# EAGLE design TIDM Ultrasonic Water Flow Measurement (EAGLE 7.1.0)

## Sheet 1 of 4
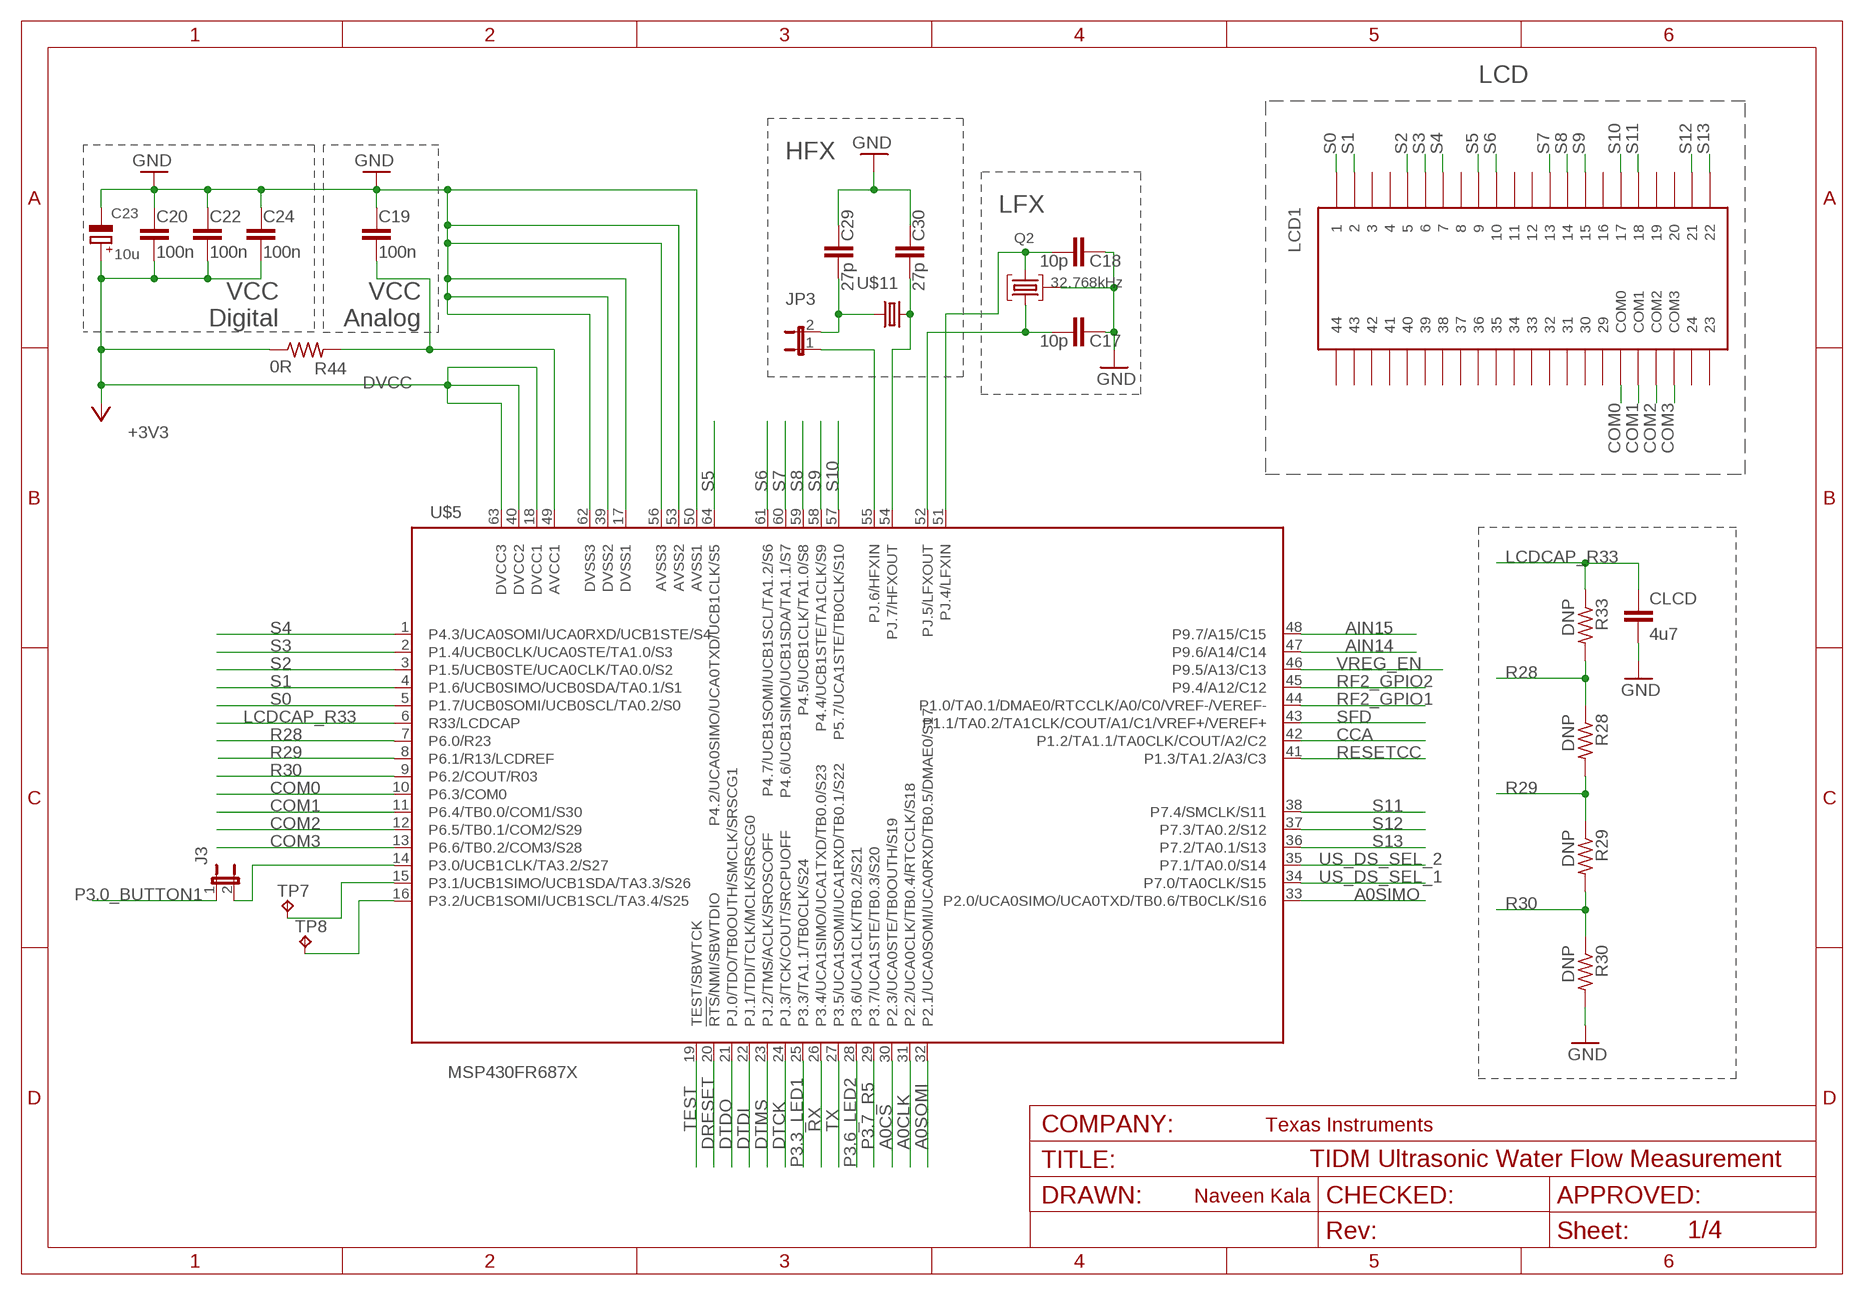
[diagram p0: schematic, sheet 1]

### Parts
C17  10p  C-EUCM0402  [0402]
C18  10p  C-EUCM0402  [0402]
C19  100n  C-EUCM0402  [0402]
C20  100n  C-EUCM0402  [0402]
C22  100n  C-EUCM0402  [0402]
C23  10u  CPOL-EUA/3216-18R  [A/3216-18R]
C24  100n  C-EUCM0402  [0402]
C29  27p  C-EUCM0402  [0402]
C30  27p  C-EUCM0402  [0402]
CLCD  4u7  CAPC0603  [0603]
J3  JP1E  [JP1]
JP3  JP1E  [JP1]
LCD1  TI_160SEG_LCD  [TI_160SEG_LCD]
Q2  32.768kHz  MS3V-T1R  [MS3V-T1R]
R28  DNP  RESR0603  [0603]
R29  DNP  RESR0603  [0603]
R30  DNP  RESR0603  [0603]
R33  DNP  RESR0603  [0603]
R44  0R  RESR0402  [0402]
TP7  TP-040  [TP-040]
TP8  TP-040  [TP-040]
U$5  MSP430FR687X  [S-PQFP-G64]
U$11  CRYSTALCTS406  [CTS406]

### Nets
A0CLK: U$5.31(P2.2/UCA0CLK/TB0.4/RTCCLK/S18) ; also sheet 2
A0CS: U$5.30(P2.3/UCA0STE/TB0OUTH/S19) ; also sheet 2
A0SIMO: U$5.33(P2.0/UCA0SIMO/UCA0TXD/TB0.6/TB0CLK/S16) ; also sheet 2,3
A0SOMI: U$5.32(P2.1/UCA0SOMI/UCA0RXD/TB0.5/DMAE0/S17) ; also sheet 2,3
AIN14: U$5.47(P9.6/A14/C14) ; also sheet 4
AIN15: U$5.48(P9.7/A15/C15) ; also sheet 4
CCA: U$5.42(P1.2/TA1.1/TA0CLK/COUT/A2/C2) ; also sheet 2
COM0: LCD1.COM0 U$5.10(P6.3/COM0)
COM1: LCD1.COM1 U$5.11(P6.4/TB0.0/COM1/S30)
COM2: LCD1.COM2 U$5.12(P6.5/TB0.1/COM2/S29)
COM3: LCD1.COM3 U$5.13(P6.6/TB0.2/COM3/S28)
DRESET: U$5.20(!RTS!/NMI/SBWTDIO) ; also sheet 3
DTCK: U$5.24(PJ.3/TCK/COUT/SRCPUOFF) ; also sheet 3
DTDI: U$5.22(PJ.1/TDI/TCLK/MCLK/SRSCG0) ; also sheet 3
DTDO: U$5.21(PJ.0/TDO/TB0OUTH/SMCLK/SRSCG1) ; also sheet 3
DTMS: U$5.23(PJ.2/TMS/ACLK/SROSCOFF) ; also sheet 3
DVCC: C20.1 C22.1 C23.+ C24.1 R44.1 U$5.18(DVCC1) U$5.40(DVCC2) U$5.63(DVCC3) ; supply symbol labelled +3V3 ; also sheet 2,3,4
GND: C17.2 C18.2 C19.2 C20.2 C22.2 C23.- C24.2 C29.2 C30.2 CLCD.2 Q2.P3(GND) R30.2 U$5.17(DVSS1) U$5.39(DVSS2) U$5.50(AVSS1) U$5.53(AVSS2) U$5.56(AVSS3) U$5.62(DVSS3) ; also sheet 2,3,4
LCDCAP_R33: CLCD.1 R33.1 U$5.6(R33/LCDCAP)
N$1: J3.2 U$5.14(P3.0/UCB1CLK/TA3.2/S27)
N$2: JP3.1 U$5.55(PJ.6/HFXIN)
N$4: TP7.1 U$5.15(P3.1/UCB1SIMO/UCB1SDA/TA3.3/S26)
N$13: C19.1 R44.2 U$5.49(AVCC1)
N$14: C30.1 U$5.54(PJ.7/HFXOUT) U$11.3
N$35: TP8.1 U$5.16(P3.2/UCB1SOMI/UCB1SCL/TA3.4/S25)
N$39: C18.1 Q2.P2 U$5.51(PJ.4/LFXIN)
N$40: C29.1 JP3.2 U$11.1
N$41: C17.1 Q2.P1 U$5.52(PJ.5/LFXOUT)
P3.0_BUTTON1: J3.1 ; also sheet 2
P3.3_LED1: U$5.25(P3.3/TA1.1/TB0CLK/S24) ; also sheet 2
P3.6_LED2: U$5.28(P3.6/UCA1CLK/TB0.2/S21) ; also sheet 2
P3.7_R5: U$5.29(P3.7/UCA1STE/TB0.3/S20) ; also sheet 4
R28: R28.1 R33.2 U$5.7(P6.0/R23)
R29: R28.2 R29.1 U$5.8(P6.1/R13/LCDREF)
R30: R29.2 R30.1 U$5.9(P6.2/COUT/R03)
RESETCC: U$5.41(P1.3/TA1.2/A3/C3) ; also sheet 2
RF2_GPIO1: U$5.44(P1.0/TA0.1/DMAE0/RTCCLK/A0/C0/VREF-/VEREF-) ; also sheet 2
RF2_GPIO2: U$5.45(P9.4/A12/C12) ; also sheet 2
RX: U$5.26(P3.4/UCA1SIMO/UCA1TXD/TB0.0/S23) ; also sheet 4
S0: LCD1.1 U$5.5(P1.7/UCB0SOMI/UCB0SCL/TA0.2/S0)
S1: LCD1.2 U$5.4(P1.6/UCB0SIMO/UCB0SDA/TA0.1/S1)
S2: LCD1.5 U$5.3(P1.5/UCB0STE/UCA0CLK/TA0.0/S2)
S3: LCD1.6 U$5.2(P1.4/UCB0CLK/UCA0STE/TA1.0/S3)
S4: LCD1.7 U$5.1(P4.3/UCA0SOMI/UCA0RXD/UCB1STE/S4)
S5: LCD1.9 U$5.64(P4.2/UCA0SIMO/UCA0TXD/UCB1CLK/S5)
S6: LCD1.10 U$5.61(P4.7/UCB1SOMI/UCB1SCL/TA1.2/S6)
S7: LCD1.13 U$5.60(P4.6/UCB1SIMO/UCB1SDA/TA1.1/S7)
S8: LCD1.14 U$5.59(P4.5/UCB1CLK/TA1.0/S8)
S9: LCD1.15 U$5.58(P4.4/UCB1STE/TA1CLK/S9)
S10: LCD1.17 U$5.57(P5.7/UCA1STE/TB0CLK/S10)
S11: LCD1.18 U$5.38(P7.4/SMCLK/S11)
S12: LCD1.21 U$5.37(P7.3/TA0.2/S12)
S13: LCD1.22 U$5.36(P7.2/TA0.1/S13)
SFD: U$5.43(P1.1/TA0.2/TA1CLK/COUT/A1/C1/VREF+/VEREF+) ; also sheet 2
TEST: U$5.19(TEST/SBWTCK) ; also sheet 3
TX: U$5.27(P3.5/UCA1SOMI/UCA1RXD/TB0.1/S22) ; also sheet 4
US_DS_SEL_1: U$5.34(P7.0/TA0CLK/S15) ; also sheet 4
US_DS_SEL_2: U$5.35(P7.1/TA0.0/S14) ; also sheet 4
VREG_EN: U$5.46(P9.5/A13/C13) ; also sheet 2
Unconnected: LCD1.3 LCD1.4 LCD1.8 LCD1.11 LCD1.12 LCD1.16 LCD1.19 LCD1.20 LCD1.23 LCD1.24 LCD1.29 LCD1.30 LCD1.31 LCD1.32 LCD1.33 LCD1.34 LCD1.35 LCD1.36 LCD1.37 LCD1.38 LCD1.39 LCD1.40 LCD1.41 LCD1.42 LCD1.43 LCD1.44

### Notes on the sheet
- LCD
- HFX
- LFX
- VCC | VCC
- Digital | Analog
- Texas Instruments
- Naveen Kala

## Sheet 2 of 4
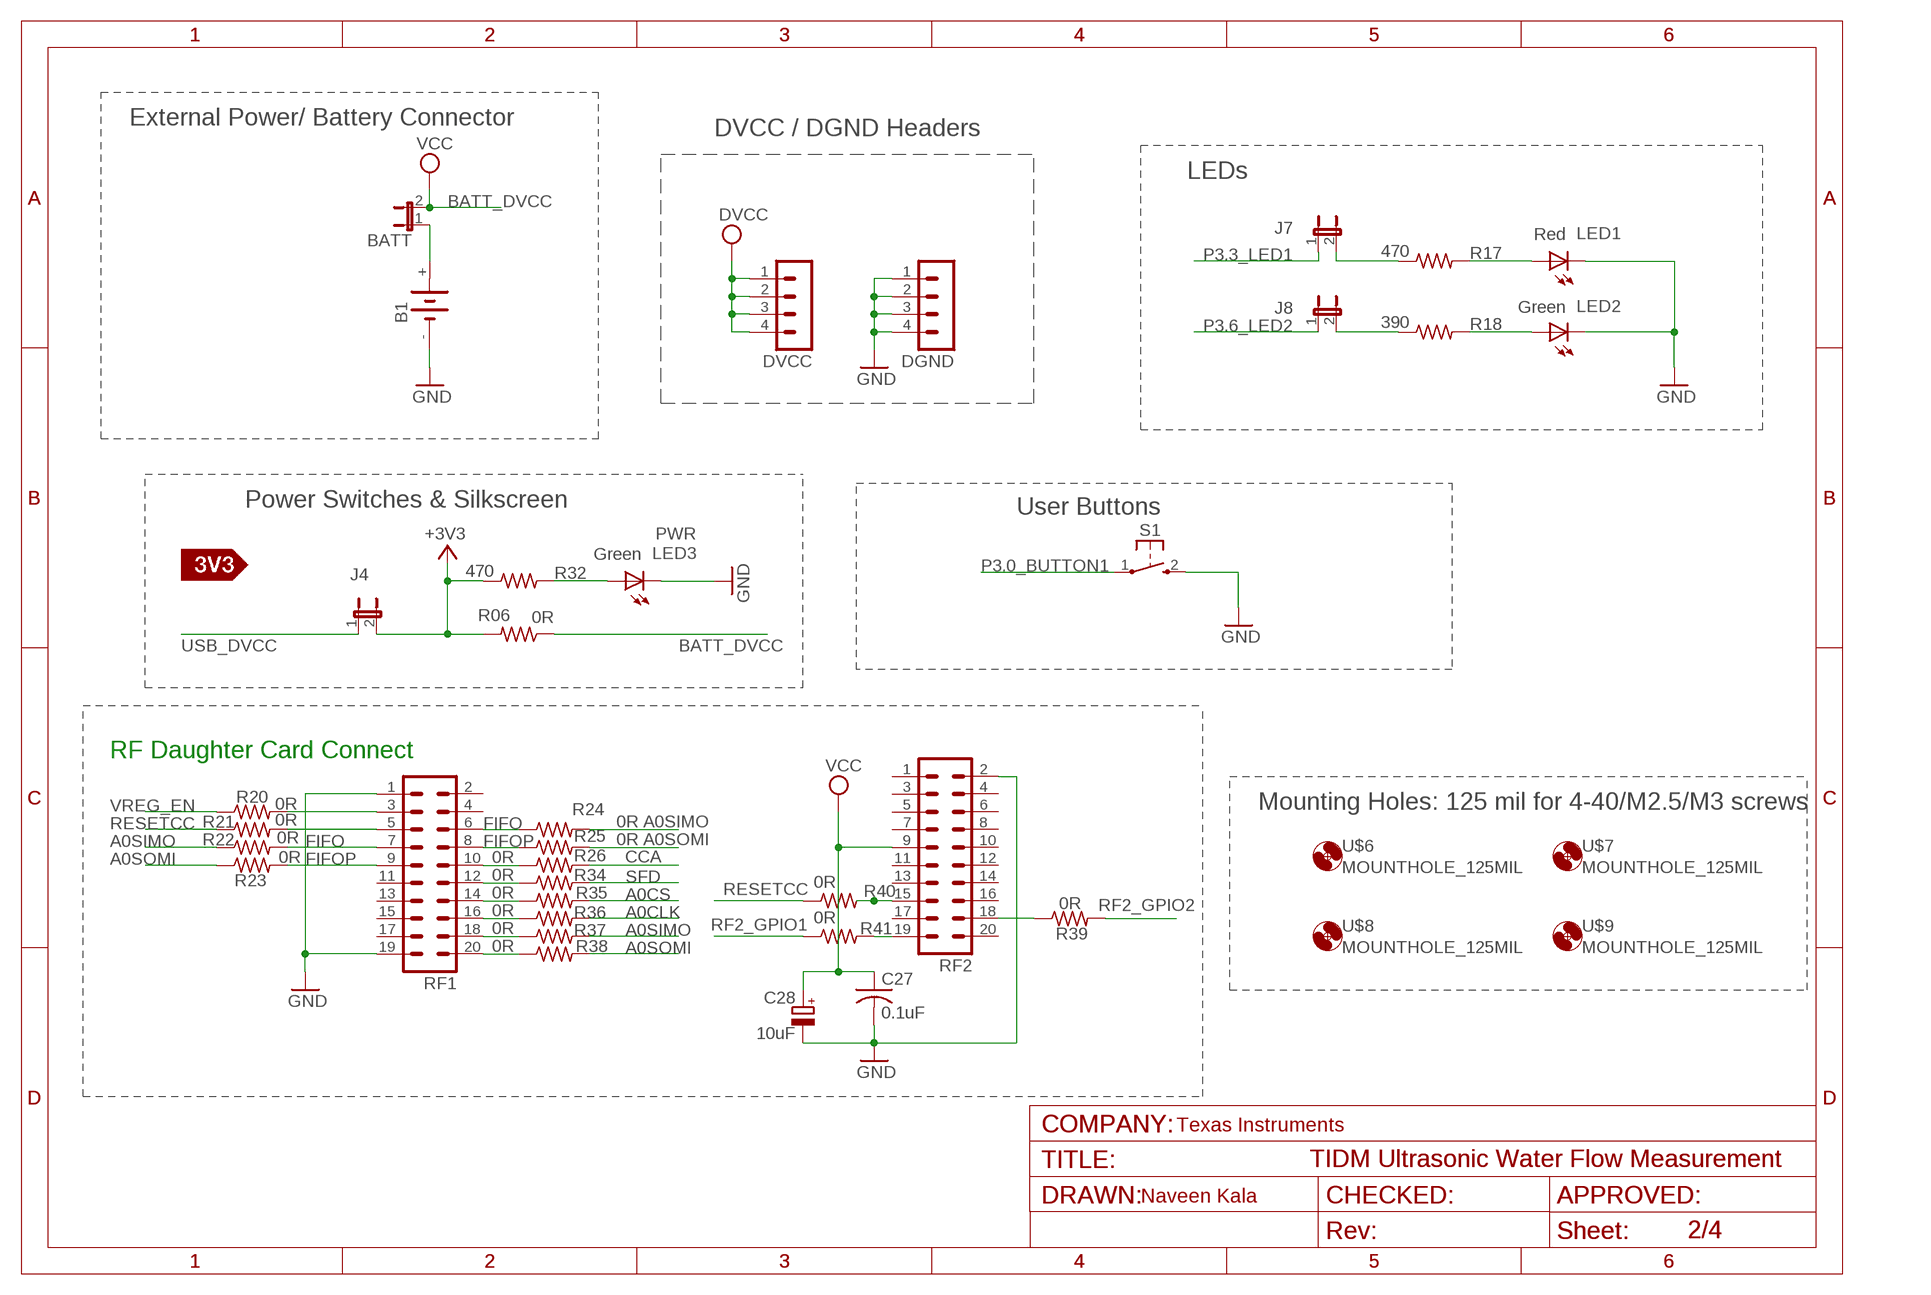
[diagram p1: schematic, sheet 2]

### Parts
B1  KS2468NO_HOLES  [KS2468_2]
BATT  JP1E  [JP1]
C27  0.1uF  C-USC0805  [C0805]
C28  10uF  CPOL-EUA/3216-18R  [A/3216-18R]
DGND  MA04-1  [MA04-1]
DVCC  MA04-1  [MA04-1]
J4  JUMPER_2.51MM  [JUMPER-2.54]
J7  JUMPER_2.51MM  [JUMPER-2.54]
J8  JUMPER_2.51MM  [JUMPER-2.54]
LED1  Red  CHIP-LED  [LED0805]
LED2  Green  CHIP-LED  [LED0805]
LED3  Green  CHIP-LED  [LED0805]
R06  0R  RESR0402  [0402]
R17  470  R-US_R0402  [R0402]
R18  390  R-US_R0402  [R0402]
R20  0R  R-US_R0603  [R0603]
R21  0R  R-US_R0603  [R0603]
R22  0R  R-US_R0603  [R0603]
R23  0R  R-US_R0603  [R0603]
R24  0R  R-US_R0603  [R0603]
R25  0R  R-US_R0603  [R0603]
R26  0R  R-US_R0603  [R0603]
R32  470  RESR0402  [0402]
R34  0R  R-US_R0603  [R0603]
R35  0R  R-US_R0603  [R0603]
R36  0R  R-US_R0603  [R0603]
R37  0R  R-US_R0603  [R0603]
R38  0R  R-US_R0603  [R0603]
R39  0R  R-US_R0603  [R0603]
R40  0R  R-US_R0603  [R0603]
R41  0R  R-US_R0603  [R0603]
RF1  TFM-110-02-SM-D-A-K  [TFM-110-02-SM-D-A-K]
RF2  TFM-110-02-SM-D-A-K  [TFM-110-02-SM-D-A-K]
S1  PB  [PBTH]
U$6  MOUNTHOLE_125MIL  [MOUNTHOLE_125MIL]
U$7  MOUNTHOLE_125MIL  [MOUNTHOLE_125MIL]
U$8  MOUNTHOLE_125MIL  [MOUNTHOLE_125MIL]
U$9  MOUNTHOLE_125MIL  [MOUNTHOLE_125MIL]
U$10  SILK_3V3_TAG  [SILK_3V3_TAG]

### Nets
$1: R20.2 RF1.3
$2: R21.2 RF1.5
A0CLK: R36.2 ; also sheet 1
A0CS: R35.2 ; also sheet 1
A0SIMO: R22.1 R24.2 R37.2 ; also sheet 1,3
A0SOMI: R23.1 R25.2 R38.2 ; also sheet 1,3
BATT_DVCC: BATT.2 R06.1 ; supply symbol labelled VCC
CCA: R26.2 ; also sheet 1
DVCC: DVCC.1 DVCC.2 DVCC.3 DVCC.4 J4.2 R06.2 R32.1 ; supply symbol labelled +3V3 ; also sheet 1,3,4
FIFO: R22.2 R24.1 RF1.6 RF1.7
FIFOP: R23.2 R25.1 RF1.8 RF1.9
GND: B1.- C27.2 C28.- DGND.1 DGND.2 DGND.3 DGND.4 LED1.C LED2.C LED3.C RF1.1 RF1.19 RF2.2 S1.2(S) ; also sheet 1,3,4
N$3: J8.2 R18.1
N$6: J7.2 R17.1
N$7: LED1.A R17.2
N$8: LED2.A R18.2
N$9: B1.+ BATT.1
N$19: R26.1 RF1.10
N$20: R34.1 RF1.12
N$23: R35.1 RF1.14
N$26: R36.1 RF1.16
N$27: R37.1 RF1.18
N$28: R38.1 RF1.20
N$29: R39.1 RF2.18
N$30: R40.2 RF2.15
N$31: R41.2 RF2.19
N$38: LED3.A R32.2
P3.0_BUTTON1: S1.1(P) ; also sheet 1
P3.3_LED1: J7.1 ; also sheet 1
P3.6_LED2: J8.1 ; also sheet 1
RESETCC: R21.1 R40.1 ; also sheet 1
RF2_GPIO1: R41.1 ; also sheet 1
RF2_GPIO2: R39.2 ; also sheet 1
SFD: R34.2 ; also sheet 1
USB_DVCC: J4.1 ; also sheet 3
VCC: C27.1 C28.+ RF2.9
VREG_EN: R20.1 ; also sheet 1
Unconnected: RF1.2 RF1.4 RF1.11 RF1.13 RF1.15 RF1.17 RF2.1 RF2.3 RF2.4 RF2.5 RF2.6 RF2.7 RF2.8 RF2.10 RF2.11 RF2.12 RF2.13 RF2.14 RF2.16 RF2.17 RF2.20

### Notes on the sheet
- External Power/ Battery Connector
- DVCC / DGND Headers
- LEDs
- Power Switches & Silkscreen
- User Buttons
- PWR
- RF Daughter Card Connect
- Mounting Holes: 125 mil for 4-40/M2.5/M3 screws
- Texas Instruments
- Naveen Kala

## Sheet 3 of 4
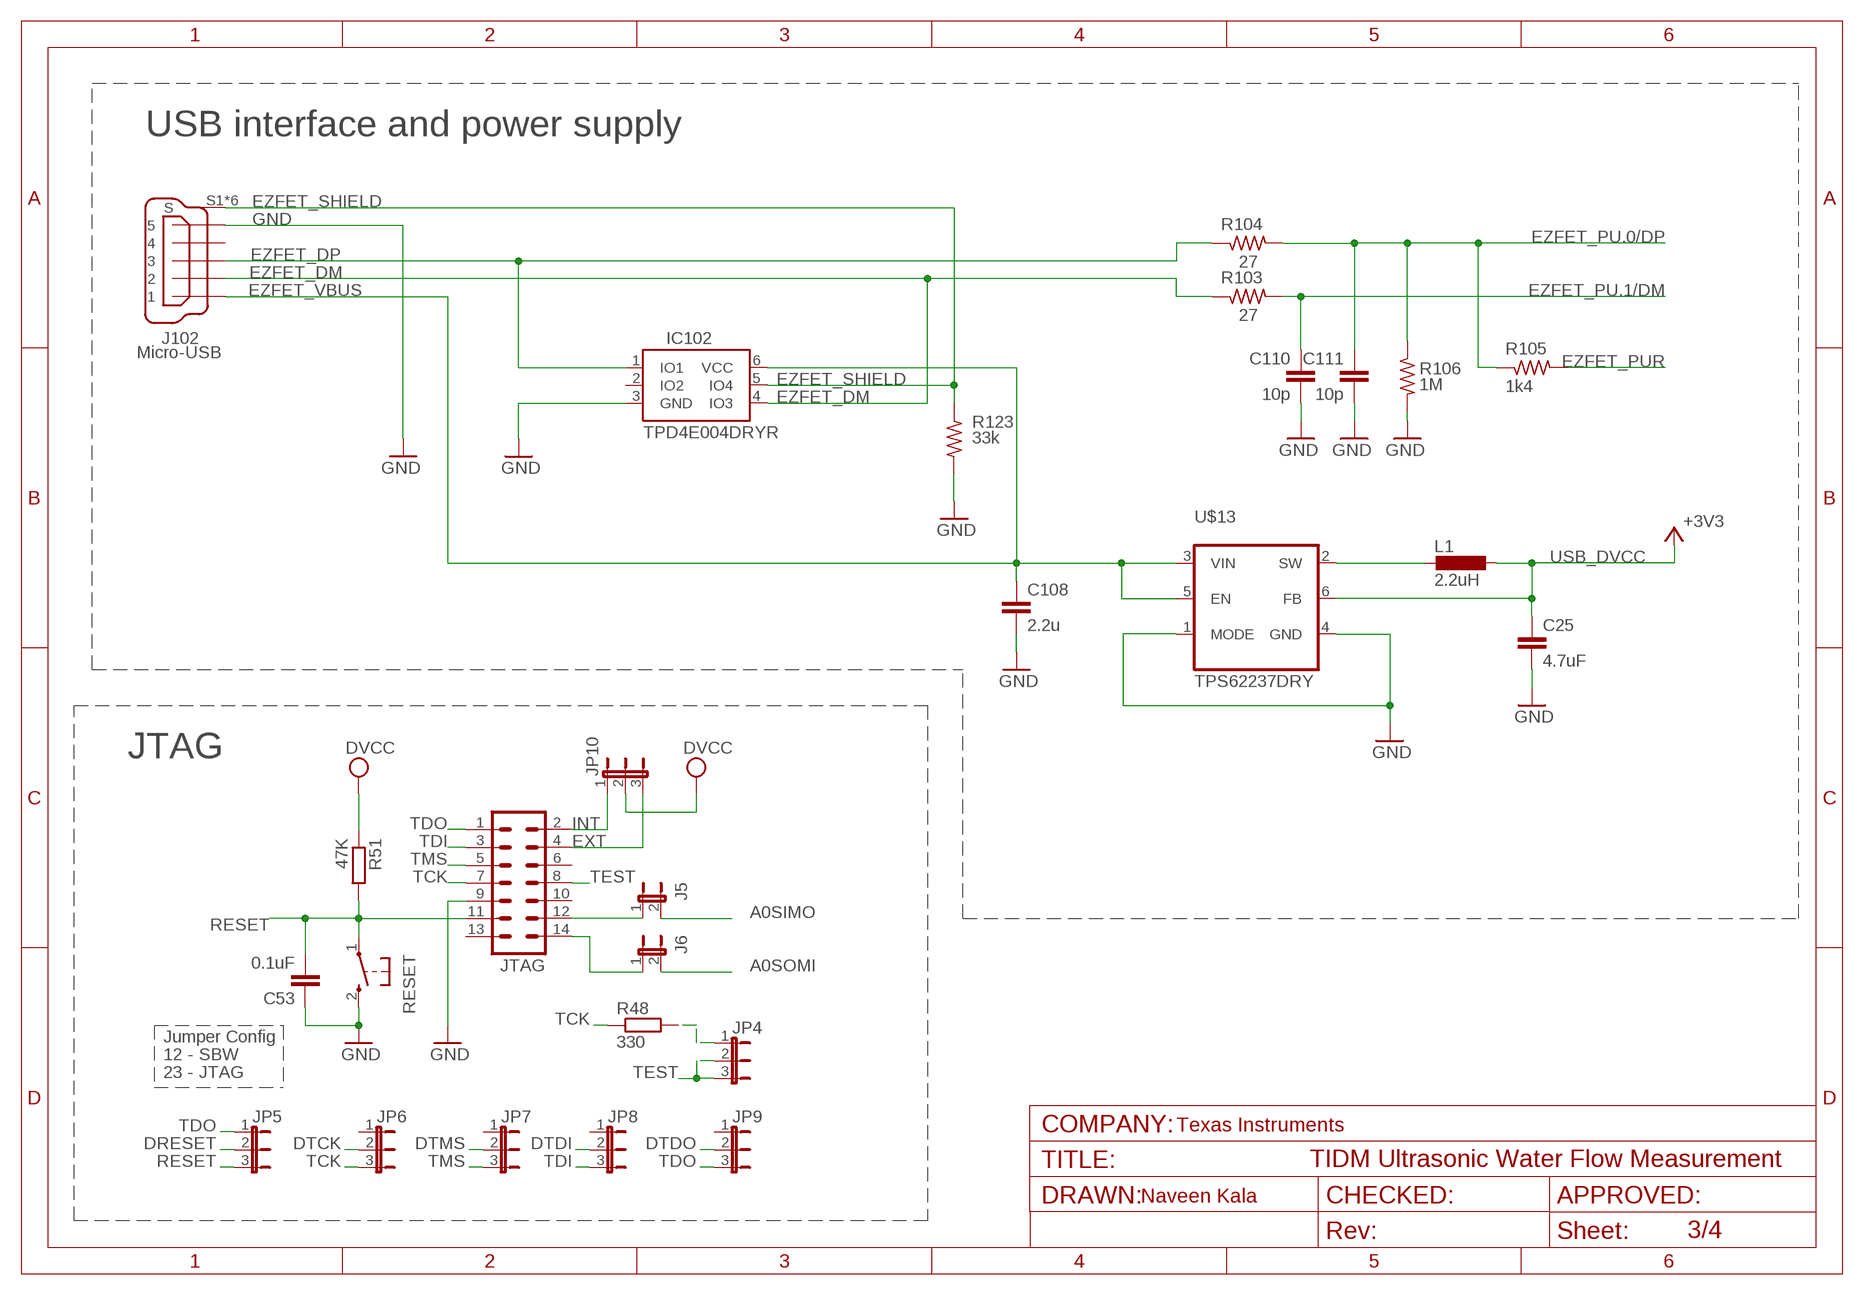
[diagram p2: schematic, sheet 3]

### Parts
C25  4.7uF  C-EUC0402  [C0402]
C53  0.1uF  C-EUC0603  [C0603]
C108  2.2u  C-EUC0603  [C0603]
C110  10p  C-EUCM0402  [0402]
C111  10p  C-EUCM0402  [0402]
IC102  TPD4E004DRYR  TPD4E004  [SON(DRY)6]
J5  JP1E  [JP1]
J6  JP1E  [JP1]
J102  Micro-USB  EZFET_MINI-USB-  [EZFET_UX62M-B-5P]
JP4  JP2E  [JP2]
JP5  JP2E  [JP2]
JP6  JP2E  [JP2]
JP7  JP2E  [JP2]
JP8  JP2E  [JP2]
JP9  JP2E  [JP2]
JP10  JP2E  [JP2]
JTAG  ML14  [ML14]
L1  2.2uH  L-EUL2012C  [L2012C]
R48  330  R-EU_R0603  [R0603]
R51  47K  R-EU_R0603  [R0603]
R103  27  RESR0402  [0402]
R104  27  RESR0402  [0402]
R105  1k4  RESR0402  [0402]
R106  1M  RESR0402  [0402]
R123  33k  RESR0402  [0402]
RESET  PB  [PBTH]
U$13  TPS62237DRY  [DRY(R-PUSON-N6)]

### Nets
A0SIMO: J5.2 ; also sheet 1,2
A0SOMI: J6.2 ; also sheet 1,2
DRESET: JP5.2 ; also sheet 1
DTCK: JP6.2 ; also sheet 1
DTDI: JP8.2 ; also sheet 1
DTDO: JP9.2 ; also sheet 1
DTMS: JP7.2 ; also sheet 1
DVCC: JP10.2 R51.1 ; also sheet 1,2,4
EXT: JP10.3 JTAG.4
EZFET_DM: IC102.4(IO3) J102.2 R103.1
EZFET_DP: IC102.1(IO1) J102.3 R104.1
EZFET_PU.0/DP: C111.1 R104.2 R105.1 R106.1
EZFET_PU.1/DM: C110.1 R103.2
EZFET_PUR: R105.2
EZFET_SHIELD: IC102.5(IO4) J102.S1(S) J102.S2(S) J102.S3(S) J102.S4(S) J102.S5(S) J102.S6(S) R123.1
EZFET_VBUS: C108.1 IC102.6(VCC) J102.1 U$13.3(VIN) U$13.5(EN)
GND: C25.2 C53.1 C108.2 C110.2 C111.2 IC102.3(GND) J102.5 JTAG.9 R106.2 R123.2 RESET.2(S) U$13.1(MODE) U$13.4(GND) ; also sheet 1,2,4
INT: JP10.1 JTAG.2
N$5: L1.2 U$13.2(SW)
N$10: JP4.1 R48.2
N$12: J6.1 JTAG.14
N$42: J5.1 JTAG.12
RESET: C53.2 JP5.3 JTAG.11 R51.2 RESET.1(P)
TCK: JP6.3 JTAG.7 R48.1
TDI: JP8.3 JTAG.3
TDO: JP5.1 JP9.3 JTAG.1
TEST: JP4.2 JP4.3 JTAG.8 ; also sheet 1
TMS: JP7.3 JTAG.5
USB_DVCC: C25.1 L1.1 U$13.6(FB) ; supply symbol labelled +3V3 ; also sheet 2
Unconnected: IC102.2(IO2) J102.4 JP6.1 JP7.1 JP8.1 JP9.1 JTAG.6 JTAG.10 JTAG.13

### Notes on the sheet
- USB interface and power supply
- JTAG
- Jumper Config
- 12 - SBW
- 23 - JTAG
- Texas Instruments
- Naveen Kala

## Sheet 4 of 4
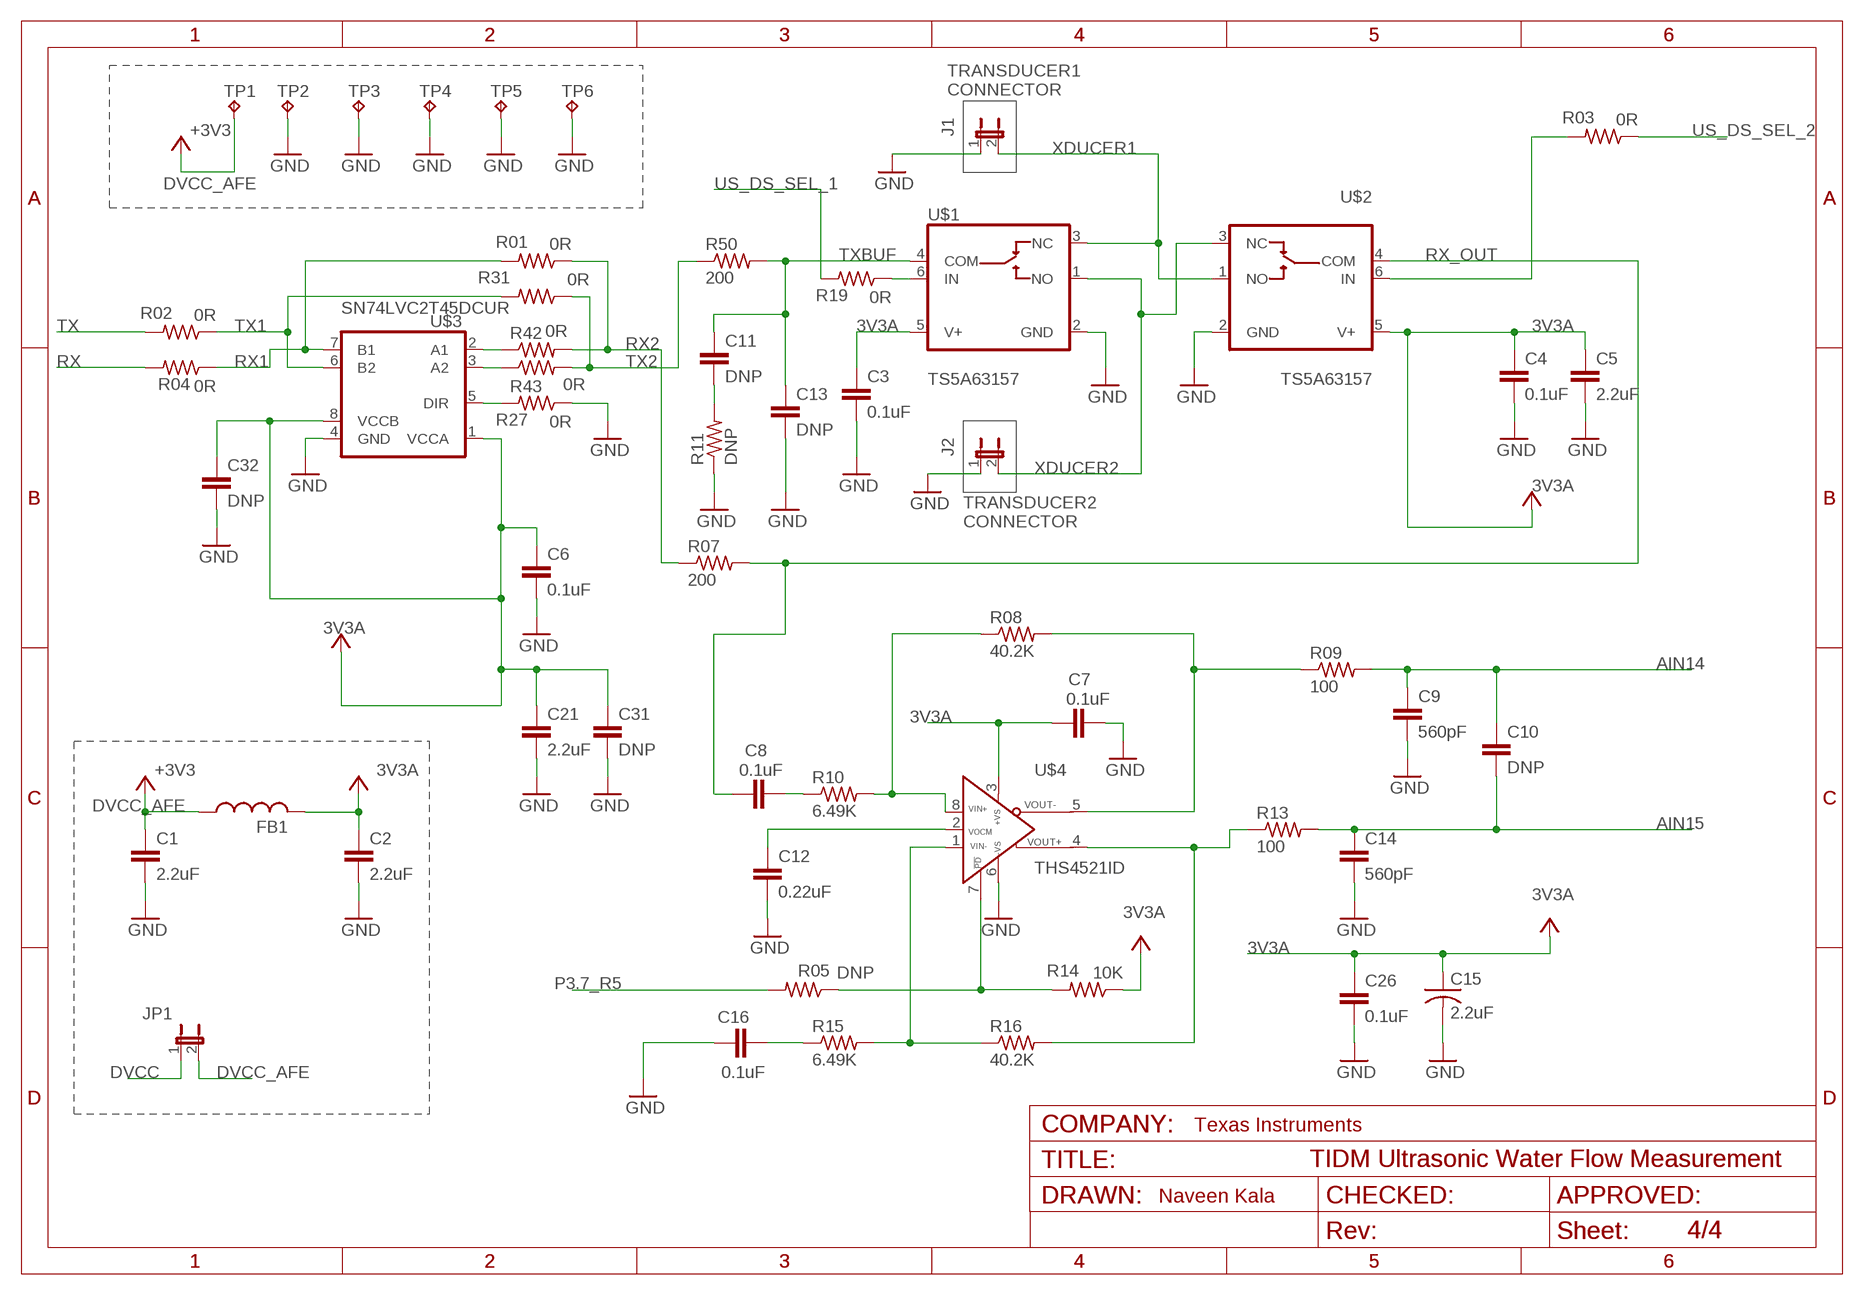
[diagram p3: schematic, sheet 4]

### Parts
C1  2.2uF  C-EUC0603  [C0603]
C2  2.2uF  C-EUC0603  [C0603]
C3  0.1uF  C-EUC0402  [C0402]
C4  0.1uF  C-EUC0402  [C0402]
C5  2.2uF  C-EUC0603  [C0603]
C6  0.1uF  C-EUC0402  [C0402]
C7  0.1uF  C-EUC0402  [C0402]
C8  0.1uF  C-EUC0603  [C0603]
C9  560pF  C-EUC0402  [C0402]
C10  DNP  C-EUC0805  [C0805@1]
C11  DNP  C-EUC0603  [C0603]
C12  0.22uF  C-EUC0402  [C0402]
C13  DNP  C-EUC0603  [C0603]
C14  560pF  C-EUC0402  [C0402]
C15  2.2uF  C-USC0603  [C0603]
C16  0.1uF  C-EUC0603  [C0603]
C21  2.2uF  C-EUC0603  [C0603]
C26  0.1uF  C-EUC0603  [C0603]
C31  DNP  C-EUC0603  [C0603]
C32  DNP  C-EUC0603  [C0603]
FB1  L-0603  [L-603]
J1  JP1E  [JP1]
J2  JP1E  [JP1]
JP1  JP1E  [JP1]
R01  0R  RESR0402  [0402]
R02  0R  RESR0402  [0402]
R03  0R  RESR0402  [0402]
R04  0R  RESR0402  [0402]
R05  DNP  RESR0402  [0402]
R07  200  R-US_R0805  [R0805]
R08  40.2K  R-US_R0805  [R0805]
R09  100  R-US_R0603  [R0603]
R10  6.49K  R-US_R0603  [R0603]
R11  DNP  R-US_R0603  [R0603]
R13  100  R-US_R0603  [R0603]
R14  10K  RESR0402  [0402]
R15  6.49K  R-US_R0603  [R0603]
R16  40.2K  R-US_R0805  [R0805]
R19  0R  RESR0402  [0402]
R27  0R  RESR0402  [0402]
R31  0R  RESR0402  [0402]
R42  0R  R-US_R0603  [R0603]
R43  0R  R-US_R0603  [R0603]
R50  200  R-US_R0805  [R0805]
TP1  TP-040  [TP-040]
TP2  TP-040  [TP-040]
TP3  TP-040  [TP-040]
TP4  TP-040  [TP-040]
TP5  TP-040  [TP-040]
TP6  TP-040  [TP-040]
U$1  TS5A63157  [DCK_R-PDSO-G6]
U$2  TS5A63157  [DCK_R-PDSO-G6]
U$3  SN74LVC2T45DCUR  [DCT(R-PDSO-G8)]
U$4  THS4521ID  [SOIC08(D-R-PDSO-G8)]

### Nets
3V3A: C2.1 C3.1 C4.1 C5.1 C6.1 C7.1 C15.1 C21.1 C26.1 C31.1 C32.1 FB1.2 R14.1 U$1.5(V+) U$2.5(V+) U$3.1(VCCA) U$3.8(VCCB) U$4.3(+VS) ; supply symbol labelled VCC
AIN14: C9.1 C10.1 R09.2 ; also sheet 1
AIN15: C10.2 C14.1 R13.2 ; also sheet 1
DIR: R27.2 U$3.5(DIR)
DVCC: JP1.1 ; also sheet 1,2,3
DVCC_AFE: C1.1 FB1.1 JP1.2 TP1.1 ; supply symbol labelled +3V3
GND: C1.2 C2.2 C3.2 C4.2 C5.2 C6.2 C7.2 C9.2 C12.2 C13.2 C14.2 C15.2 C16.1 C21.2 C26.2 C31.2 C32.2 J1.1 J2.1 R11.1 R27.1 TP2.1 TP3.1 TP4.1 TP5.1 TP6.1 U$1.2(GND) U$2.2(GND) U$3.4(GND) U$4.6(-VS) ; also sheet 1,2,3
N$11: R19.1 U$1.6(IN)
N$15: C11.2 R11.2
N$16: R03.2 U$2.6(IN)
N$17: R08.2 R09.1 U$4.5(VOUT-)
N$18: R13.1 R16.2 U$4.4(VOUT+)
N$21: R15.2 R16.1 U$4.1(VIN-)
N$22: C16.2 R15.1
N$24: R08.1 R10.2 U$4.8(VIN+)
N$25: C8.2 R10.1
N$32: R05.1 R14.2 U$4.7(!PD!)
N$33: R42.1 U$3.2(A1)
N$34: R43.1 U$3.3(A2)
P3.7_R5: R05.2 ; also sheet 1
RX: R04.2 ; also sheet 1
RX1: R01.2 R04.1 U$3.7(B1)
RX2: R01.1 R07.1 R42.2
RX_OUT: C8.1 R07.2 U$2.4(COM)
TX: R02.2 ; also sheet 1
TX1: R02.1 R31.2 U$3.6(B2)
TX2: R31.1 R43.2 R50.1
TXBUF: C11.1 C13.1 R50.2 U$1.4(COM)
US_DS_SEL_1: R19.2 ; also sheet 1
US_DS_SEL_2: R03.1 ; also sheet 1
VOCM: C12.1 U$4.2(VOCM)
XDUCER1: J1.2 U$1.3(NC) U$2.1(NO)
XDUCER2: J2.2 U$1.1(NO) U$2.3(NC)

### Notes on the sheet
- TRANSDUCER1
  CONNECTOR
- 3V3A
- TRANSDUCER2
  CONNECTOR
- 3V3A
- 3V3A
- 3V3A
- 3V3A
- Texas Instruments
- Naveen Kala

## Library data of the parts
B1 = _MSP430:KS2468
BATT J1-J3 J5 J6 JP1 JP3 = jumper:JP1E: JUMPER
C1-C14 C16-C22 C24-C26 C29-C32 C108 C110 C111 = rcl:C-EU: CAPACITOR, European symbol
C15 C27 = rcl:C-US: CAPACITOR, American symbol
C23 C28 = rcl:CPOL-EU: POLARIZED CAPACITOR, European symbol
C53 = resistor:C-EU: CAPACITOR, European symbol
CLCD = MSP430_CapResistor:CAP
DGND DVCC = custom_con-lstb:MA04-1: PIN HEADER; OC_FARNELL: unknown; OC_NEWARK: unknown
FB1 = HVK-Ultrasonic-FM:L-0603
IC102 = eZFET:TPD4E004
J4 J7 J8 = launchpad:JUMPER_2.51MM
J102 = MSP-EXP430G6021:EZFET_MINI-USB-: MINI USB Connector Source: http://www.hirose.co.jp/cataloge_hp/e24000019.pdf
JP4-JP10 = custom_jumper:JP2E: JUMPER
JTAG = con-ml:ML14: HARTING; OC_FARNELL: unknown; OC_NEWARK: unknown
L1 = rcl:L-EU: INDUCTOR, European symbol
LCD1 = Personal:TI_160SEG_LCD
LED1-LED3 = launchpad:CHIP-LED
Q2 = microcrystal:MS3V-T1R
R01-R06 R14 R19 R27-R33 R44 R103-R106 R123 = CapResistor:RES
R07-R09 R10 R11 R13 R15-R18 R20-R26 R34-R43 R50 = rcl:R-US_: RESISTOR, American symbol
R48 R51 = resistor:R-EU_: RESISTOR, European symbol
RESET S1 = electricalmeter:PB: OMRON SWITCH
RF1 RF2 = _MSP430:TFM-110-02-SM-D-A-K
TP1-TP8 = keystone:TP: TEST POINT
U$1 U$2 = HVK-Ultrasonic-FM:TS5A63157
U$3 = HVK-Ultrasonic-FM:SN74LVC2T45DCUR
U$4 = HVK-Ultrasonic-FM:THS4521ID
U$5 = HVK-Ultrasonic-FM:MSP430FR687X
U$6-U$9 = MSP-EXP432:MOUNTHOLE_125MIL
U$10 = MSP-EXP432:SILK_3V3_TAG
U$11 = crystal:CRYSTAL: CRYSTAL; OC_FARNELL: unknown; OC_NEWARK: unknown
U$13 = HVK-Ultrasonic-FM:TPS62237DRY

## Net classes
2 Power: width 0.203 mm, drill 0.305 mm, clearance 0.152 mm to class 0, clearance 0.152 mm to class 1, clearance 0.152 mm

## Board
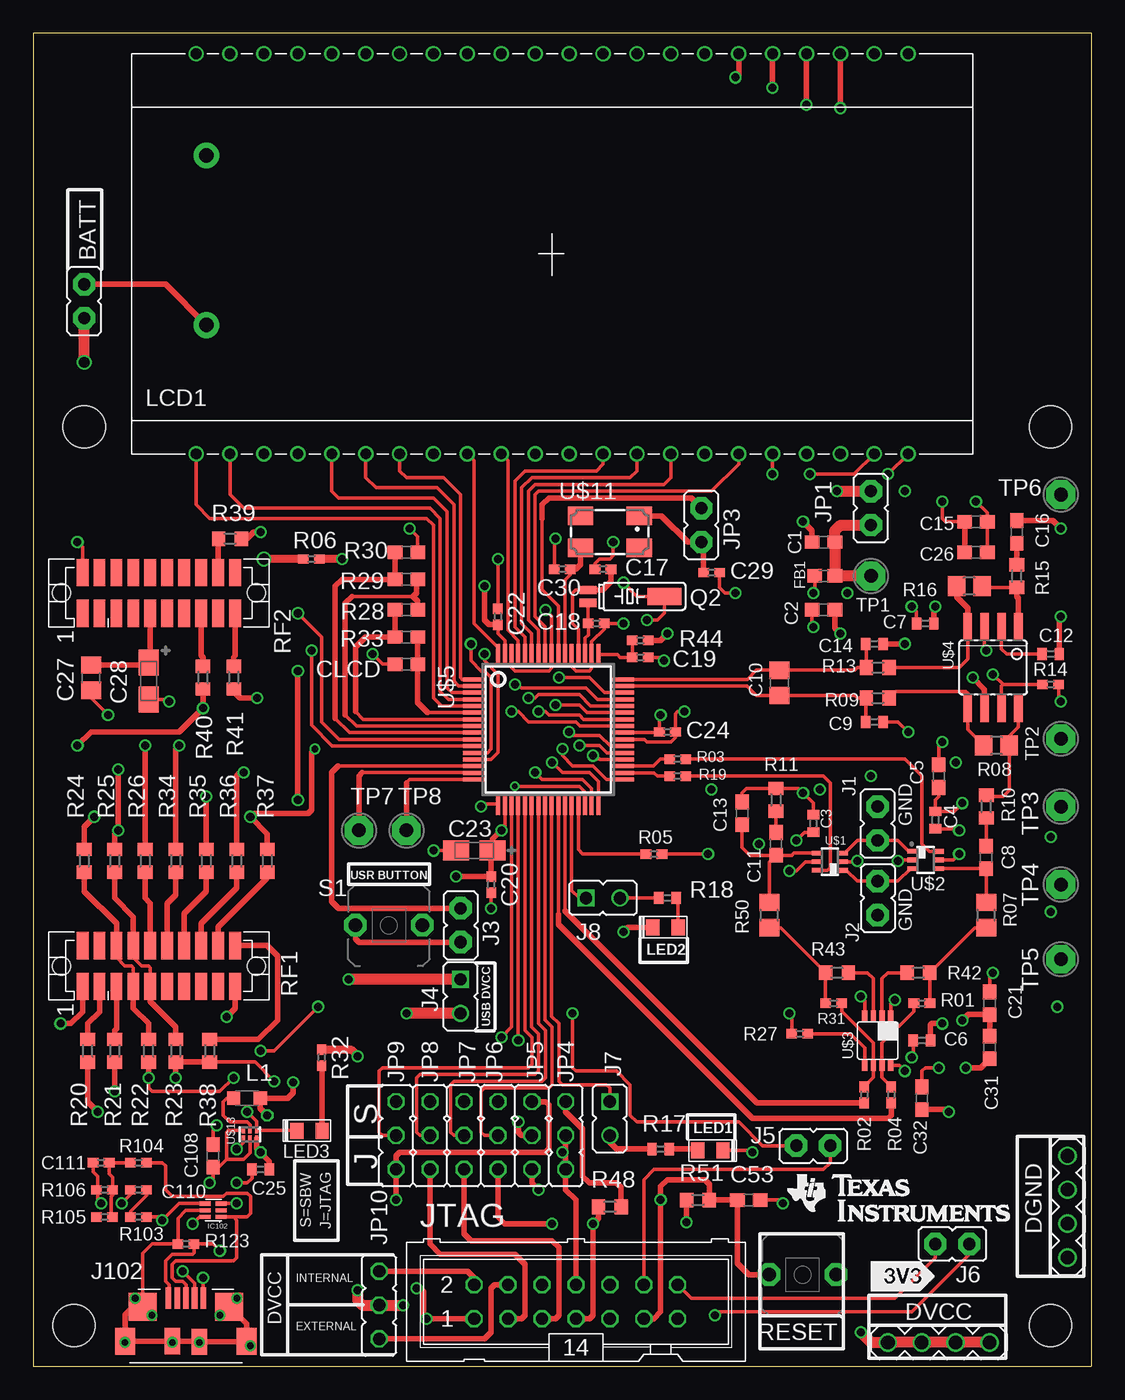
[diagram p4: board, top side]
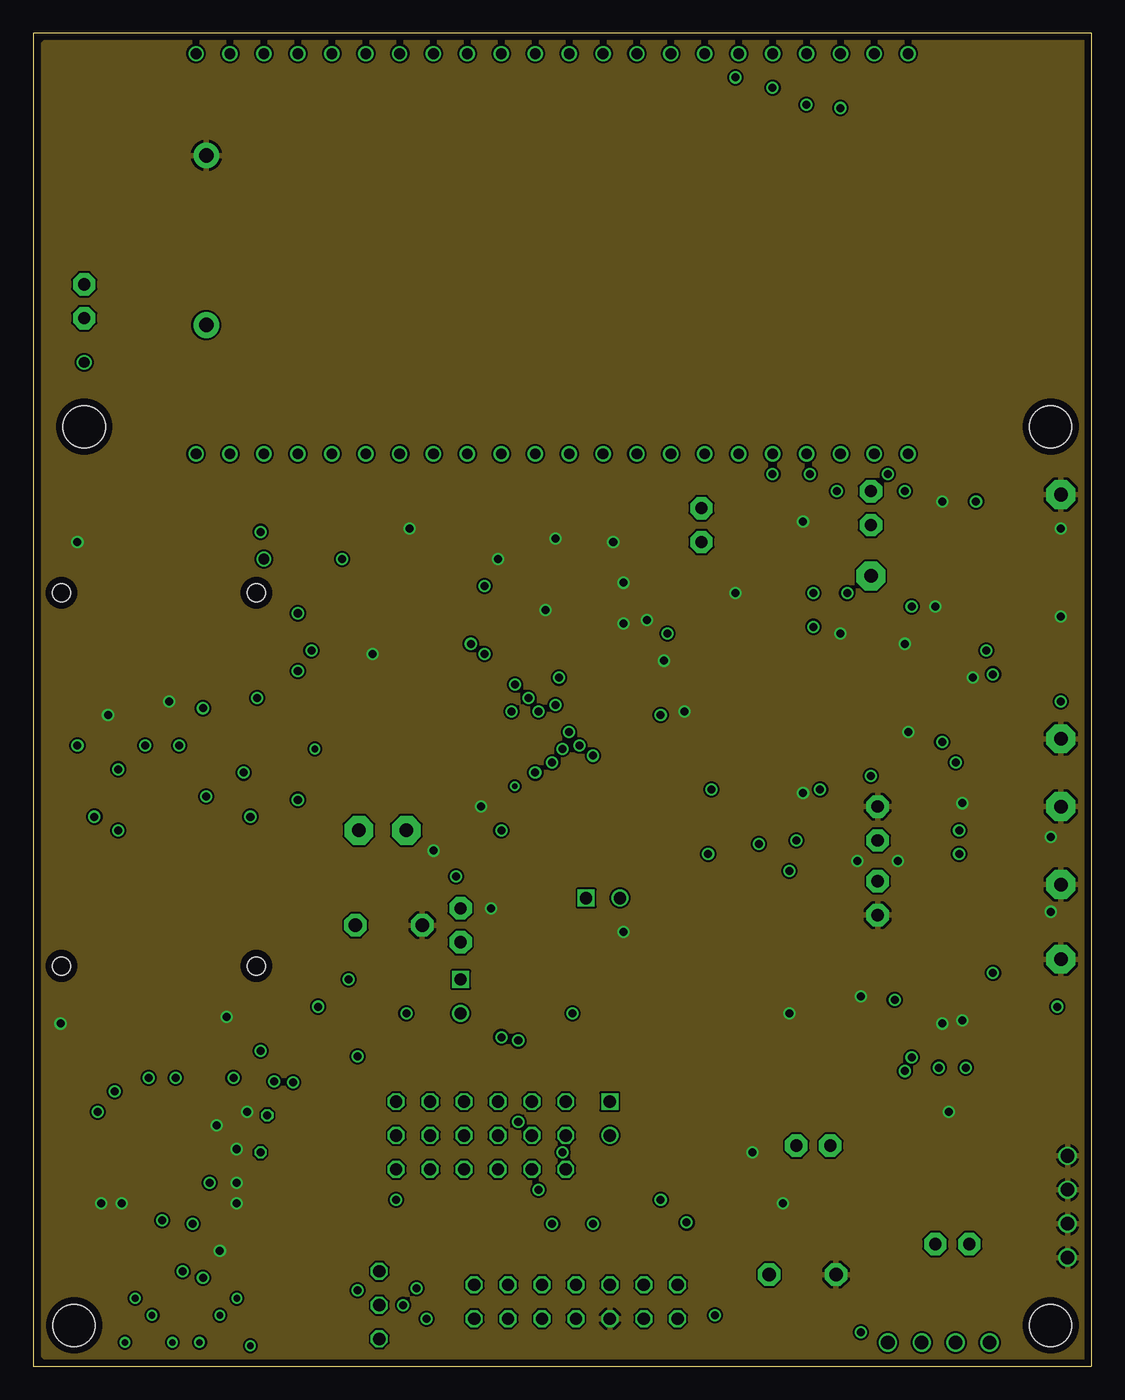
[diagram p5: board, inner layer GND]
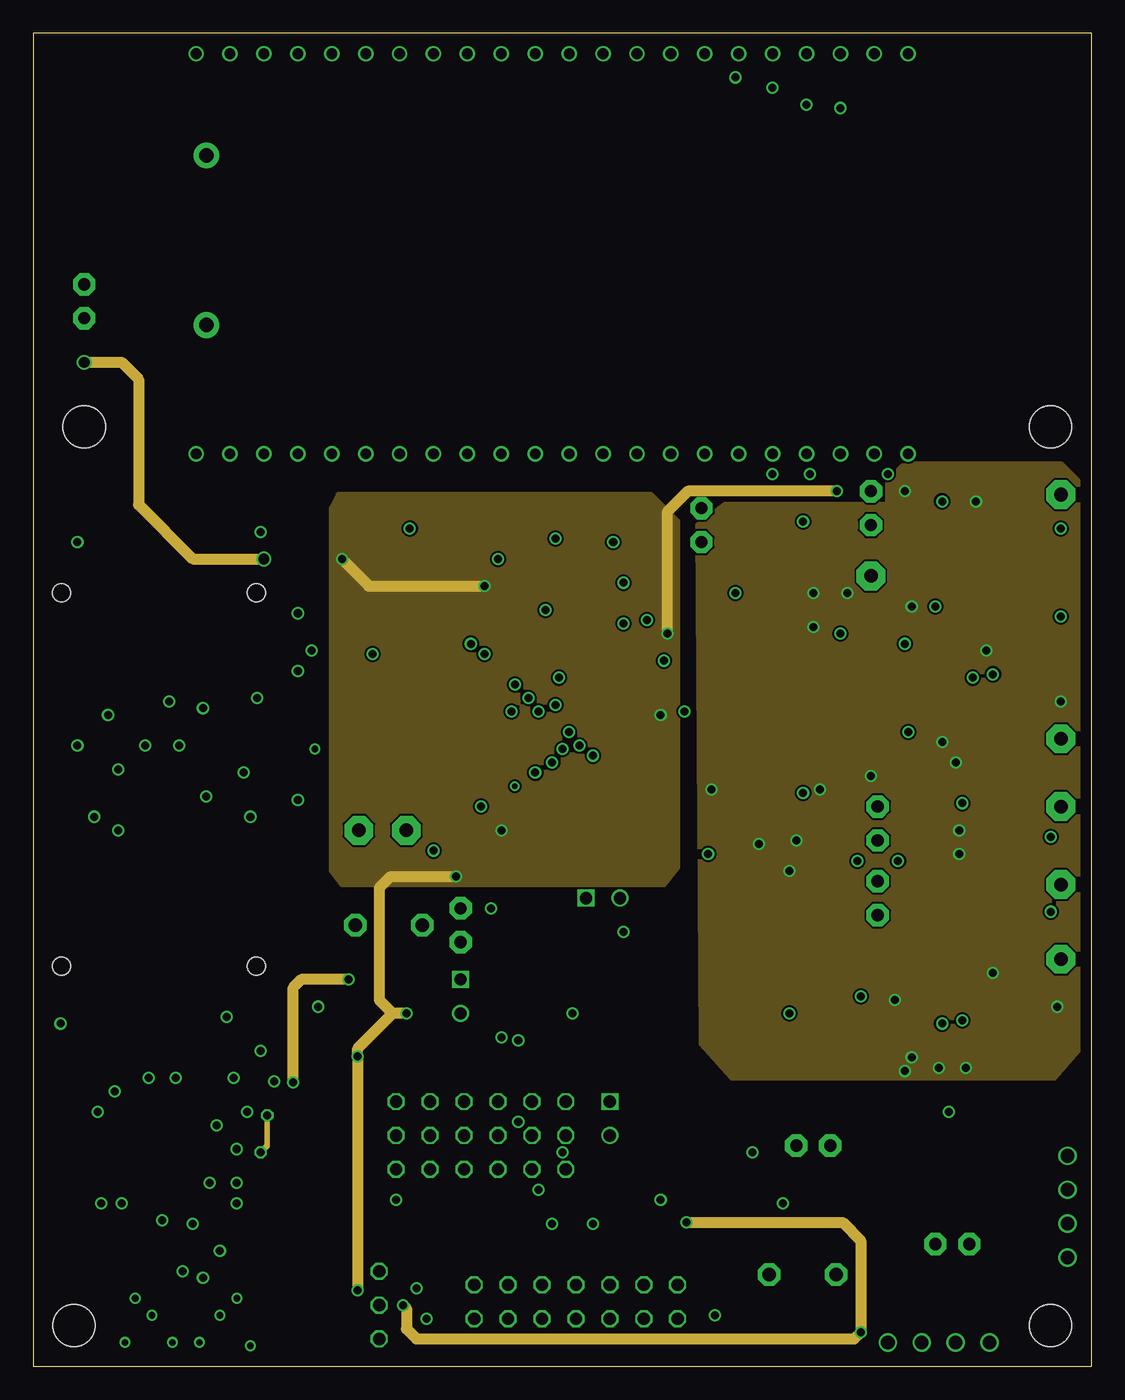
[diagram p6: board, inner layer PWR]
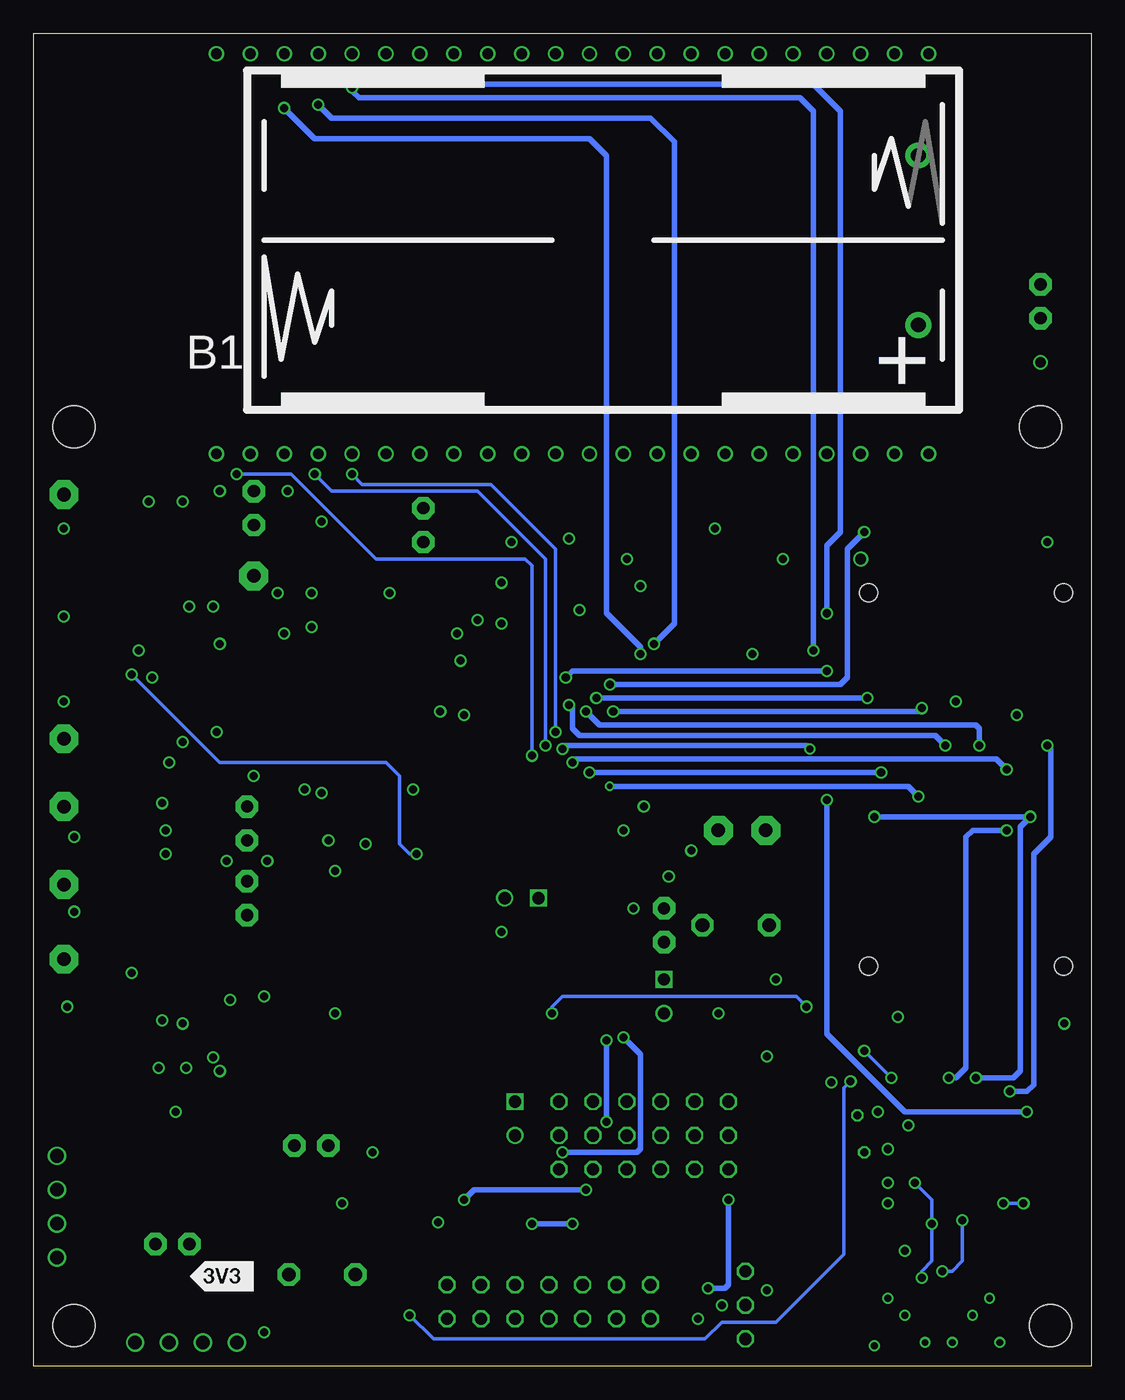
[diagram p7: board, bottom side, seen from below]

Size 79.25 x 99.82 mm. Coordinates in mm from the lower left corner, seen from the top.
Outline: 0,0 79.25,0 79.25,99.82 0,99.82 0,0
Copper layers (1+2*15+16): Top 0.0178mm / dielectric 12mil / GND 0.0356mm / dielectric 27mil / PWR 0.0356mm / dielectric 12mil / Bottom 0.0178mm
Design rules "5529 Design Rules": minimum track width 6mil, minimum drill 12mil, track to track 6mil, track to pad 6mil, pad to pad 6mil, via to via 6mil, smd to smd 6mil, copper to edge 20mil, drill to drill 8mil, minimum pad ring 7mil, minimum via ring 6mil, stop-mask expansion 0mil, vias tented up to drill 25mil, thermal gap 8mil

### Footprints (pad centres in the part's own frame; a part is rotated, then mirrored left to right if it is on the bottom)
KS2468_2 = drill 1.1 pad 1.93: + 24.892,-6.35; - 24.892,6.35
JP1 = drill 0.914 pad 1.676 octagon: 1 0,-1.27; 2 0,1.27
C0603 = smd 1.1 x 1: 1 -0.85,0; 2 0.85,0
C0402 = smd 0.7 x 0.9: 1 -0.65,0; 2 0.65,0
C0805@1 = smd 1.3 x 1.5: 1 -0.95,0; 2 0.95,0
0402 = smd 0.8 x 0.7: 1 -0.6,0; 2 0.6,0
A/3216-18R = smd 1.95 x 1.5: + 1.375,0; - -1.375,0
C0805 = smd 1.3 x 1.5: 1 -0.95,0; 2 0.95,0
0603 = smd 1.1 x 1: 1 -0.85,0; 2 0.85,0
MA04-1 = drill 1.016: 1 -3.81,0; 2 -1.27,0; 3 1.27,0; 4 3.81,0
L-603 = smd 1.1 x 1: 1 -0.85,0; 2 0.65,0
SON(DRY)6 = smd 0.81 x 0.305: 1 -0.1,0; 2 -0.1,-0.5; 3 -0.1,-1; 4 1.1,-1; 5 1.1,-0.5; 6 1.1,0
JUMPER-2.54 = drill 0.914 square: 1 0,-1.27 | drill 0.914: 2 0,1.27
EZFET_UX62M-B-5P = smd 0.42 x 1.6: 1 1.3,1.3; 2 0.65,1.3; 3 0,1.3; 4 -0.65,1.3; 5 -1.3,1.3 | smd 2.1 x 2.1: S1 -3.25,0.65; S2 3.25,0.65 | smd 1.5 x 2: S3 -4.55,-1.95; S4 4.55,-1.95 | smd 1.144 x 1.949: S5 -1.016,-1.93; S6 1.016,-1.981
JP2 = drill 0.914 octagon: 1 -2.54,0; 2 0,0; 3 2.54,0
ML14 = drill 0.914 octagon: 1 -7.62,-1.27; 2 -7.62,1.27; 3 -5.08,-1.27; 4 -5.08,1.27; 5 -2.54,-1.27; 6 -2.54,1.27; 7 0,-1.27; 8 0,1.27; 9 2.54,-1.27; 10 2.54,1.27; 11 5.08,-1.27; 12 5.08,1.27; 13 7.62,-1.27; 14 7.62,1.27
L2012C = smd 1 x 1: 1 -1,0; 2 1,0
TI_160SEG_LCD = drill 0.8: 1 4.826,0; 2 7.366,0; 3 9.906,0; 4 12.446,0; 5 14.986,0; 6 17.526,0; 7 20.066,0; 8 22.606,0; 9 25.146,0; 10 27.686,0; 11 30.226,0; 12 32.766,0; 13 35.306,0; 14 37.846,0; 15 40.386,0; 16 42.926,0; 17 45.466,0; 18 48.006,0; 19 50.546,0; 20 53.086,0; 21 55.626,0; 22 58.166,0; 23 58.166,29.972; 24 55.626,29.972; 29 42.926,29.972; 30 40.386,29.972; 31 37.846,29.972; 32 35.306,29.972; 33 32.766,29.972; 34 30.226,29.972; 35 27.686,29.972; 36 25.146,29.972; 37 22.606,29.972; 38 20.066,29.972; 39 17.526,29.972; 40 14.986,29.972; 41 12.446,29.972; 42 9.906,29.972; 43 7.366,29.972; 44 4.826,29.972; COM0 45.466,29.972; COM1 48.006,29.972; COM2 50.546,29.972; COM3 53.086,29.972
LED0805 = smd 1 x 1.2: A 1.052,0.102; C -0.848,0.102
MS3V-T1R = smd 0.635 x 1.27: P1 -0.47,-4.43; P2 0.47,-4.43 | smd 1.27 x 2.54: P3 0,1.3
R0805 = smd 1.3 x 1.5: 1 -0.95,0; 2 0.95,0
R0603 = smd 1 x 1.1: 1 -0.85,0; 2 0.85,0
R0402 = smd 0.7 x 0.9: 1 -0.65,0; 2 0.65,0
PBTH = drill 1.016 pad 1.676 octagon: 1 -0.001,0.001; 2 5.001,0.001
TFM-110-02-SM-D-A-K = smd 2.032 x 0.889: 1 -1.524,5.715; 2 1.524,5.715; 3 -1.524,4.445; 4 1.524,4.445; 5 -1.524,3.175; 6 1.524,3.175; 7 -1.524,1.905; 8 1.524,1.905; 9 -1.524,0.635; 10 1.524,0.635; 11 -1.524,-0.635; 12 1.524,-0.635; 13 -1.524,-1.905; 14 1.524,-1.905; 15 -1.524,-3.175; 16 1.524,-3.175; 17 -1.524,-4.445; 18 1.524,-4.445; 19 -1.524,-5.715; 20 1.524,-5.715 | hole 1.359: 0,7.303; 0,-7.303
TP-040 = drill 1.016 pad 2.159 octagon: 1 0,0
DCK_R-PDSO-G6 = smd 0.35 x 0.8: 1 -0.97,-0.92; 2 -0.32,-0.92; 3 0.33,-0.92; 4 0.33,0.98; 5 -0.32,0.98; 6 -0.96,0.98
DCT(R-PDSO-G8) = smd 0.4 x 0.8: 1 -0.975,-1.875; 2 -0.325,-1.875; 3 0.325,-1.875; 4 0.975,-1.875; 5 0.975,1.875; 6 0.325,1.875; 7 -0.325,1.875; 8 -0.975,1.875
SOIC08(D-R-PDSO-G8) = smd 0.66 x 2.032: 1 -1.905,-3.835; 2 -0.635,-3.835; 3 0.635,-3.835; 4 1.905,-3.835; 5 1.905,2.311; 6 0.635,2.311; 7 -0.635,2.311; 8 -1.905,2.311
S-PQFP-G64 = smd 0.3 x 1.6: 1 -3.69,-5.13; 2 -3.19,-5.13; 3 -2.69,-5.13; 4 -2.19,-5.13; 5 -1.69,-5.13; 6 -1.19,-5.13; 7 -0.69,-5.13; 8 -0.19,-5.13; 9 0.31,-5.13; 10 0.81,-5.13; 11 1.31,-5.13; 12 1.81,-5.13; 13 2.31,-5.13; 14 2.81,-5.13; 15 3.31,-5.13; 16 3.81,-5.13; 33 3.81,6.07; 34 3.31,6.07; 35 2.81,6.07; 36 2.31,6.07; 37 1.81,6.07; 38 1.31,6.07; 39 0.81,6.07; 40 0.31,6.07; 41 -0.19,6.07; 42 -0.69,6.07; 43 -1.19,6.07; 44 -1.69,6.07; 45 -2.19,6.07; 46 -2.69,6.07; 47 -3.19,6.07; 48 -3.69,6.07 | smd 1.6 x 0.3: 17 5.66,-3.28; 18 5.66,-2.78; 19 5.66,-2.28; 20 5.66,-1.78; 21 5.66,-1.28; 22 5.66,-0.78; 23 5.66,-0.28; 24 5.66,0.22; 25 5.66,0.72; 26 5.66,1.22; 27 5.66,1.72; 28 5.66,2.22; 29 5.66,2.72; 30 5.66,3.22; 31 5.66,3.72; 32 5.66,4.22; 49 -5.54,4.22; 50 -5.54,3.72; 51 -5.54,3.22; 52 -5.54,2.72; 53 -5.54,2.22; 54 -5.54,1.72; 55 -5.54,1.22; 56 -5.54,0.72; 57 -5.54,0.22; 58 -5.54,-0.28; 59 -5.54,-0.78; 60 -5.54,-1.28; 61 -5.54,-1.78; 62 -5.54,-2.28; 63 -5.54,-2.78; 64 -5.54,-3.28
MOUNTHOLE_125MIL = hole 3.175: 0,0
CTS406 = smd 1.9 x 1.4: 1 -2.2,-1.2; 2 2.2,-1.2; 3 2.2,1.2; 4 -2.2,1.2
DRY(R-PUSON-N6) = smd 0.25 x 0.45: 1 -0.72,-0.12; 2 -0.22,-0.12; 3 0.28,-0.12; 4 0.28,0.45; 5 -0.22,0.45; 6 -0.72,0.45

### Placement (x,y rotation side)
B1  37.85,84.33 0 bottom
BATT  3.81,79.76 180 top
C1  59.18,61.72 180 top
C2  59.18,56.64 0 top
C3  58.42,40.64 90 top
C4  67.56,40.89 90 top
C5  67.82,44.2 270 top
C6  66.55,24.38 0 top
C7  66.8,55.63 0 top
C8  71.37,38.1 90 top
C9  62.99,48.26 0 top
C10  55.88,51.18 90 top
C11  55.63,39.12 90 top
C12  76.2,53.34 0 top
C13  53.09,41.4 90 top
C14  62.99,54.1 0 top
C15  70.61,63.25 180 top
C16  73.66,62.48 270 top
C17  42.67,59.69 180 top
C18  42.16,55.63 0 top
C19  45.47,53.09 0 top
C20  34.29,36.07 270 top
C21  71.63,27.18 270 top
C22  34.8,56.13 90 top
C23  33.02,38.61 0 top
C24  47.5,47.5 0 top
C25  17.02,14.73 180 top
C26  70.61,60.96 180 top
C27  4.32,51.56 270 top
C28  8.64,51.31 90 top
C29  50.8,59.44 0 top
C30  39.62,59.69 180 top
C31  71.63,23.88 90 top
C32  66.55,20.07 270 top
C53  53.59,12.45 180 top
C108  13.46,15.75 90 top
C110  7.87,13.21 180 top
C111  5.08,15.24 180 top
CLCD  27.94,52.58 180 top
DGND  77.47,11.94 90 top
DVCC  67.82,1.78 0 top
FB1  59.18,59.18 180 top
IC102  13.97,11.18 180 top
J1  63.25,40.64 180 top
J2  63.25,35.05 0 top
J3  32,33.02 0 top
J4  32,27.69 180 top
J5  58.42,16.51 90 top
J6  68.83,9.14 270 top
J7  43.18,18.54 180 top
J8  42.67,35.05 270 top
J102  11.43,3.81 0 top
JP1  62.74,64.26 180 top
JP3  50.04,62.99 180 top
JP4  39.88,17.27 270 top
JP5  37.34,17.27 270 top
JP6  34.8,17.27 270 top
JP7  32.26,17.27 270 top
JP8  29.72,17.27 270 top
JP9  27.18,17.27 270 top
JP10  25.91,4.57 270 top
JTAG  40.64,4.83 0 top
L1  16,20.07 180 top
LCD1  7.37,68.33 0 top
LED1  50.8,16.26 180 top
LED2  47.24,32.77 0 top
LED3  20.57,17.53 0 top
Q2  45.97,57.66 270 top
R01  66.55,27.18 180 top
R02  62.23,20.32 270 top
R03  48.26,45.47 0 top
R04  64.26,20.32 270 top
R05  46.48,38.35 180 top
R06  20.83,60.45 0 top
R07  71.37,33.78 90 top
R08  72.14,46.48 180 top
R09  63.25,50.04 180 top
R10  71.37,41.91 90 top
R11  55.63,42.42 270 top
R13  63.25,52.32 180 top
R14  76.2,51.05 180 top
R15  73.66,59.18 270 top
R16  70.1,58.42 180 top
R17  46.99,16.26 0 top
R18  47.5,35.05 0 top
R19  48.26,44.2 180 top
R20  4.06,23.62 90 top
R21  6.1,23.62 90 top
R22  8.64,23.62 90 top
R23  10.67,23.62 90 top
R24  3.81,37.85 90 top
R25  6.1,37.85 90 top
R26  8.38,37.85 90 top
R27  57.4,24.89 0 top
R28  27.94,56.64 0 top
R29  27.94,58.93 180 top
R30  27.94,60.96 0 top
R31  59.94,27.18 0 top
R32  21.59,23.11 270 top
R33  27.94,54.61 180 top
R34  10.67,37.85 90 top
R35  12.95,37.85 90 top
R36  15.24,37.85 90 top
R37  17.53,37.85 90 top
R38  13.21,23.62 270 top
R39  14.73,61.98 0 top
R40  12.71,51.56 90 top
R41  15.02,51.56 90 top
R42  66.29,29.46 0 top
R43  60.2,29.46 180 top
R44  45.47,54.36 180 top
R48  43.18,11.94 0 top
R50  55.12,33.78 90 top
R51  49.78,12.45 0 top
R103  7.87,11.18 180 top
R104  7.87,15.24 180 top
R105  5.33,11.18 180 top
R106  5.33,13.21 180 top
R123  11.43,9.14 0 top
RESET  55.12,6.86 0 top
RF1  9.4,29.97 90 top
RF2  9.4,57.91 90 top
S1  24.13,33.02 0 top
TP1  62.74,59.18 270 top
TP2  76.96,46.99 90 top
TP3  76.96,41.91 90 top
TP4  76.96,36.07 90 top
TP5  76.96,30.48 270 top
TP6  76.96,65.28 90 top
TP7  24.38,40.13 0 top
TP8  27.94,40.13 0 top
U$1  59.69,38.1 90 top
U$2  66.8,37.59 270 top
U$3  63.25,24.38 180 top
U$4  71.88,51.56 180 top
U$5  38.1,47.75 270 top
U$6  3.05,3.05 0 top
U$7  3.81,70.36 0 top
U$8  76.2,70.36 0 top
U$9  76.2,3.05 0 top
U$10  62.74,5.59 0 top
U$11  43.18,62.48 180 top
U$12  [LOGO16_TPLACE]  56.39,10.67 0 top
U$13  16,17.53 180 top

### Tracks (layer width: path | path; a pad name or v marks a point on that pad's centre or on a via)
3V3A  (via drill 0.6)
  Top 0.254: v70.61,64.77 71.46,63.92 C15.1 C26.1 | FB1.2 58.53,58.02 v58.42,57.91 | C2.1 58.33,55.46 v58.42,55.37 | U$4.3 71.25,53.72 v71.37,53.59 | C7.1 66.15,56.53 v65.79,56.9 | U$1.5 57.85,37.78 57.15,37.08 v56.64,37.08 | R14.1 76.8,49.95 v76.96,49.78 | C3.1 57.77,39.99 v57.15,39.37 | U$2.5 68.9,37.91 v69.34,38.35 | C4.1 69.23,40.24 v69.34,40.13 | C5.1 67.82,46.48 v68.07,46.74 | U$3.1 64.22,27.14 v64.52,27.43 | C21.1 71.63,29.21 v71.88,29.46 | U$3.8 64.87,22.51 v65.28,22.1 | C6.1 65.9,23.23 v65.79,23.11 | C32.1 66.55,22.1 66.8,22.35 v67.82,22.35
  Top 0.406: v69.85,22.35 70.95,22.35 C31.1
  other vias: 65.28,65.53 60.96,57.91 58.93,43.18 62.74,44.2 50.8,43.18 76.71,26.92 54.36,39.12 69.09,45.21
  pour PWR: 50.04,24.13 52.32,21.59 76.45,21.59 78.23,23.62 78.23,66.29 76.96,67.56 65.28,67.56 64.01,66.29 64.01,64.52 51.82,64.52 49.78,62.99
$1
  Top 0.406: RF1.3 4.95,26.54 4.06,25.65 R20.2
$2
  Top 0.406: RF1.5 6.22,25.27 6.1,25.15 R21.2
A0CLK  (via drill 0.6)
  Top 0.254: 37.85,44.2 v37.59,44.45 38.1,43.94 41.15,43.94 41.82,43.27 U$5.31
  Top 0.406: v15.75,44.45 15.49,44.45 15.24,44.2 R36.2
  Bottom 0.406: v37.59,44.45 v15.75,44.45
A0CS  (via drill 0.41, 0.6)
  Top 0.254: U$5.30 41.32,43.01 40.89,43.43 v36.07,43.43
  Top 0.406: v12.95,42.67 R35.2
  Bottom 0.406: v36.07,43.43 13.72,43.43 v12.95,42.67
A0SIMO  (via drill 0.5, 0.6)
  Top 0.254: U$5.33 42.93,43.94 41.91,44.96 40.39,44.96 39.62,45.72 v39.62,46.23 | J5.2 54.61,16.51 52.83,18.29 45.21,18.29 44.7,18.8 44.7,21.08 43.69,22.1 40.64,22.1 40.39,22.35 v40.39,26.42 | v8.64,21.59 8.64,20.83 8.89,20.57 13.97,20.57 v14.99,21.59 | v17.02,23.62 18.03,23.62 v21.34,26.92
  Top 0.406: R24.2 3.81,40.39 v4.57,41.15 | R22.1 v8.64,21.59 | R37.2 17.53,39.88 v16.26,41.15 16.51,41.4 20.57,41.4 20.83,41.66 20.83,45.97 v21.08,46.23
  Bottom 0.254: 40.13,26.67 v40.39,26.42 40.39,26.92 39.62,27.69 22.1,27.69 v21.34,26.92 | v14.99,21.59 v17.02,23.62
  Bottom 0.406: v39.62,46.23 39.37,46.48 21.34,46.48 v21.08,46.23 | v16.26,41.15 v4.57,41.15 5.33,40.39 5.33,22.1 5.84,21.59 v8.64,21.59
A0SOMI  (via drill 0.6)
  Top 0.254: v38.86,45.21 39.62,44.45 41.66,44.45 42.32,43.79 U$5.32 | v18.03,21.34 16.6,22.77 R38.2 | J6.2 70.1,8.38 65.79,4.06 51.31,4.06 v51.05,3.81
  Top 0.406: R38.2 R23.1 v10.67,21.59 | R25.2 6.1,39.88 v6.35,40.13 v6.35,44.7
  Bottom 0.254: v18.03,21.34 18.54,20.83 18.54,8.38 23.62,3.3 27.69,3.3 28.96,2.03 49.28,2.03 v51.05,3.81
  Bottom 0.406: v6.35,40.13 8.89,40.13 9.4,39.62 9.4,22.35 10.16,21.59 v10.67,21.59 | v38.86,45.21 38.61,45.47 7.11,45.47 v6.35,44.7
AIN14
  Top 0.254: U$5.47 53.45,50.94 54.16,50.23 C10.1 61.53,50.23 61.72,50.04 R09.2 62.34,49.98 C9.1
AIN15
  Top 0.254: U$5.48 53.47,51.44 54.16,52.13 C10.2 61.53,52.13 61.72,52.32 R13.2 62.4,54.05 C14.1
BATT_DVCC  (via drill 0.8)
  Top 0.61: R06.1 v17.27,60.45
  Top 0.813: v3.81,75.18 BATT.2
  PWR 0.813: 17.02,60.45 v17.27,60.45 11.94,60.45 7.87,64.52 7.87,73.91 6.6,75.18 v3.81,75.18
CCA  (via drill 0.6)
  Top 0.254: U$5.42 41.22,48.44 40.89,48.77 38.61,48.77 38.35,49.02 v37.85,49.02
  Top 0.406: v8.38,46.48 R26.2
  Bottom 0.406: v8.38,46.48 8.38,47.75 8.64,48.01 36.83,48.01 v37.85,49.02
COM0  (via drill 0.6)
  Top 0.254: U$5.10 22.91,46.94 21.59,48.26 21.59,54.61 v19.81,56.39
  Top 0.406: v52.58,96.52 52.83,96.77 LCD1.COM0
  Bottom 0.406: v52.58,96.52 52.07,96.01 20.83,96.01 18.8,93.98 18.8,62.48 19.81,61.47 v19.81,56.39
COM1  (via drill 0.6)
  Top 0.254: U$5.11 22.39,46.44 20.83,48.01 v20.83,53.59
  Top 0.406: v55.37,95.76 LCD1.COM1
  Bottom 0.254: 20.83,60.71 20.83,61.21
  Bottom 0.406: v20.83,53.59 20.83,60.71 20.83,93.98 21.84,95 54.86,95 55.37,95.5 v55.37,95.76
COM2  (via drill 0.6)
  Top 0.254: U$5.12 34,45.94 34.29,46.23 34.29,51.56 33.78,52.07 33.53,52.07 32.77,52.83 v32.77,54.1
  Top 0.406: v57.91,94.49 LCD1.COM2
  Bottom 0.406: v57.91,94.49 56.9,93.47 33.02,93.47 31.24,91.69 31.24,55.63 v32.77,54.1
COM3  (via drill 0.6)
  Top 0.254: U$5.13 34.27,45.44 34.8,45.97 34.8,51.82 33.78,52.83 v33.78,53.34
  Top 0.406: v60.45,94.23 LCD1.COM3
  Bottom 0.406: v60.45,94.23 58.17,91.95 37.59,91.95 36.32,90.68 36.32,56.39 33.78,53.85 v33.78,53.34
DIR
  Top 0.254: U$3.5 62.27,23.84 61.21,24.89 R27.2
DRESET  (via drill 0.6)
  Top 0.254: U$5.20 v36.32,24.39 v36.32,24.38
  Top 0.406: v36.32,18.29 36.32,17.53 36.58,17.27 JP5.2
  Bottom 0.406: v36.32,24.38 v36.32,18.29
DTCK
  Top 0.254: U$5.24 38.32,25.94 38.86,25.4 38.86,21.08 38.61,20.83 33.78,20.83 33.53,20.57 33.53,17.53 33.78,17.27 JP6.2
DTDI
  Top 0.254: U$5.22 37.32,25.42 37.85,24.89 37.85,22.1 37.59,21.84 28.96,21.84 28.7,21.59 28.7,17.53 28.96,17.27 JP8.2
DTDO
  Top 0.254: U$5.21 36.83,25.15 37.34,24.64 37.34,22.61 37.08,22.35 26.16,22.35 25.91,22.1 25.91,17.53 26.16,17.27 JP9.2
DTMS
  Top 0.254: U$5.23 37.82,25.68 38.35,25.15 38.35,21.59 38.1,21.34 31.5,21.34 31.24,21.08 31.24,17.53 31.5,17.27 JP7.2
DVCC  (via drill 0.6)
  Top 0.254: U$5.40 46.84,47.44 C24.1 46.9,48.68 v46.99,48.77 | 34.29,38.5 C23.+ | U$5.63 35.32,54.34 34.8,54.86 C22.1 | U$5.18 35.32,40.4 v35.05,40.13
  Top 0.406: 34.29,38.5 C20.1 v31.66,36.67 | C23.+ 34.4,39.48 v35.05,40.13 | R44.1 46.99,54.36 v47.5,54.86 | C22.1 34.13,55.53 33.78,55.88 v33.78,58.42 | R51.1 v48.93,10.76
  Top 0.61: v23.11,60.45 R06.2 | R32.1 23.78,23.71 v24.3,23.2
  Top 0.813: DVCC.4 DVCC.3 DVCC.2 DVCC.1 62.74,1.78 v61.98,2.54 | v60.2,65.53 JP1.1 | J4.2 v27.94,26.42 | v24.3,5.68 24.3,4.91 24.64,4.57 JP10.2 v27.69,4.57
  PWR 0.813: v47.5,54.86 47.5,64.01 49.02,65.53 v60.2,65.53 | v23.11,60.45 25.15,58.42 v33.78,58.42 | v31.66,36.67 26.76,36.67 25.91,35.81 25.91,27.43 26.92,26.42 | v27.94,26.42 26.92,26.42 | v24.3,5.68 v24.3,23.2 24.3,23.79 26.92,26.42 | v48.93,10.76 60.62,10.76 61.98,9.4 v61.98,2.54 61.47,2.03 28.7,2.03 27.94,2.79 27.94,4.32 v27.69,4.57
  pour PWR: 22.35,64.26 22.35,37.08 23.11,36.07 47.24,36.07 48.26,37.34 48.26,63.25 46.23,65.28 22.86,65.28
DVCC_AFE
  Top 0.813: 59.94,61.81 C1.1 | C1.1 FB1.1 TP1.1 | C1.1 60.03,62.57 60.45,62.99 JP1.2
EXT
  Top 0.406: JTAG.4 34.54,6.1 34.29,5.84 34.29,2.54 33.78,2.03 JP10.3
EZFET_DM  (via drill 0.6)
  Top 0.254: J102.2 12.08,6.21 v11.18,7.11 | R103.1 9.4,11.18 v9.65,10.92 10.91,12.18 IC102.4
  Bottom 0.254: v9.65,10.92 9.65,7.87 10.41,7.11 v11.18,7.11
EZFET_DP
  Top 0.254: J102.3 11.43,6.1 11.18,6.35 10.67,6.35 10.41,6.6 10.41,7.62 10.67,7.87 14.99,7.87 15.24,8.13 15.24,10.92 14.99,11.18 | IC102.1 14.99,11.18 | R104.1 9.65,15.24 9.91,14.99 9.91,13.21 10.41,12.7 14.22,12.7 14.48,12.95 16,12.95 16.26,12.7 16.26,11.43 16,11.18 14.99,11.18
EZFET_PU.0/DP
  Top 0.254: R104.2 C111.1 5.68,14.39 5.93,14.13 R106.1 5.93,12.79 5.84,12.7 5.84,11.27 R105.1
EZFET_PU.1/DM
  Top 0.254: C110.1 8.47,12.79 7.27,11.59 R103.2
EZFET_SHIELD  (via drill 0.5)
  Top 0.254: J102.S1 8.18,8.43 8.89,9.14 R123.1 10.83,11.08 11.42,11.68 IC102.5
  Top 0.406: 10.39,1.86 J102.S5 | J102.S2 15.98,3.16 J102.S4 | v12.45,1.78 J102.S6 | J102.S3 6.88,3.83 7.37,4.32 | 7.37,4.32 8.04,4.32 J102.S1 8.24,4.46 v8.89,3.81 | J102.S5 6.9,1.88 J102.S3 | J102.S5 12.39,1.88 J102.S6 | J102.S6 15.95,1.83 J102.S4 | J102.S3 6.88,1.8 v6.86,1.78 | 7.37,4.32 7.37,4.83 v7.62,5.08 | J102.S2 14.68,4.52 v15.24,5.08 | J102.S4 15.98,1.8 v16.26,1.52 | v10.41,1.78 J102.S5 | v13.97,3.81 14.03,3.81 J102.S2
EZFET_VBUS  (via drill 0.6)
  Top 0.254: 16.22,16.48 U$13.5 16.22,15.97 15.75,15.49 14.48,15.49 | U$13.3 14.6,17.65 14.48,17.53 14.48,15.49 | IC102.6 12.45,11.18 v11.94,10.67 | J102.1 12.73,6.57 v12.7,6.6 | v13.21,13.72 13.46,13.97 C108.1 13.88,14.9 14.48,15.49
  Bottom 0.254: v13.21,13.72 11.94,12.45 v11.94,10.67 11.94,7.87 12.7,7.11 v12.7,6.6
FIFO
  Top 0.254: RF1.7 7.49,29.84 7.37,29.97 6.86,29.97 6.22,30.61 RF1.6
  Top 0.406: R24.1 3.81,35.56 6.22,33.15 RF1.6 | RF1.7 7.49,26.8 8.64,25.65 R22.2
FIFOP
  Top 0.254: RF1.8 7.49,30.61 8.13,29.97 8.64,29.97 8.76,29.84 RF1.9
  Top 0.406: R25.1 6.1,35.05 7.49,33.66 RF1.8 | RF1.9 8.76,27.3 10.67,25.4 R23.2
GND  (via drill 0.6)
  Top 0.254: J102.5 10.16,5.14 10.16,6.1 9.91,6.35 9.91,7.87 10.41,8.38 11.94,8.38 12.03,8.47 R123.2 13.46,9.14 v13.97,8.64 | C111.2 4.48,14.57 4.83,14.22 4.83,13.3 R106.2 4.83,13.12 4.83,12.45 v5.08,12.19 | v6.6,12.19 7.27,12.86 C110.2 | IC102.3 15.22,12.18 v15.24,12.19 | C108.2 13.46,17.78 v13.72,18.03 | U$3.4 62.27,27.39 v61.98,27.69 | U$5.39 45.77,46.94 45.97,46.74 47.75,46.74 48.1,47.08 C24.2 48.1,48.86 48.26,49.02 v48.77,49.02 | v38.35,56.64 38.82,56.18 U$5.56 38.82,52.28 38.61,52.07 36.07,52.07 35.82,52.32 U$5.62 | U$5.53 40.32,52.39 40.64,52.07 41.66,52.07 41.82,52.23 U$5.50 41.82,54.27 42.76,55.21 C18.2 v44.2,55.63 | 19.46,17.63 LED3.C 19.71,17.65 U$13.1 16.72,18.33 v16,19.05 | C5.2 67.82,42.67 67.56,42.42 C4.2 68.98,41.54 v69.6,42.16 | U$2.2 64.84,37.91 v64.77,37.85 | R27.1 56.8,26.25 v56.64,26.42 | C13.2 53.09,42.93 53.43,43.27 R11.1 57.32,43.27 v57.66,42.93 58.42,42.16 C3.2 | U$1.2 61.66,37.78 v61.72,37.85 | C15.2 68.33,63.25 68.07,63.5 v68.07,64.77 | LED1.C 53.7,16.15 v53.85,16 | C53.1 55.88,12.45 v56.13,12.19 | C29.2 51.4,58.33 51.82,57.91 v52.58,57.91 | v45.97,55.88 46.74,55.88 47.27,56.42 Q2.P3 45.21,57.66 v44.2,58.67 | C22.2 v34.8,60.45 | C30.2 39.02,61.88 v39.12,61.98 | C27.2 4.32,50.04 v5.59,48.77 | C28.- 10.01,49.93 v10.16,49.78 | C19.2 46.99,53.09 v47.24,52.83 | RF2.2 3.68,61.34 v3.3,61.72 | CLCD.2 26.16,52.58 v25.4,53.34 | C23.- v29.97,38.61 | U$5.17 33.71,42.09 v33.53,41.91 | C20.2 v34.29,34.29 | U$13.4 15.72,16.74 v15.24,16.26 | R30.2 28.79,62.14 v28.19,62.74 | C25.2 16.37,14.08 16,13.72 v15.24,13.72 | C9.2 64.77,48.26 v65.53,47.5 | C17.2 42.07,60.11 42.42,60.45 43.18,60.45 43.43,60.71 v43.43,61.72
  Top 0.406: 59.94,56.55 C2.2 60.03,55.28 v60.45,54.86 | RF1.19 15.11,26.8 v14.48,26.16 | LED2.C 44.55,32.87 v44.2,32.51 | C31.2 C21.2 70.02,26.33 v69.6,25.91 | C6.2 67.2,25.54 67.31,25.65 v68.07,25.65 | C32.2 68.41,19.22 v68.58,19.05 | U$4.6 71.25,50.67 v70.36,51.56 | C15.2 C26.2 | C16.1 76.37,63.33 v76.96,62.74 | C7.2 67.45,56.78 v67.56,56.9 | C1.2 58.33,62.57 v57.66,63.25 | C12.2 76.85,56.02 v76.96,56.13 | C14.2 v65.28,54.1 | RF1.1 3.68,26.54 2.79,25.65 v2.03,25.65
  Bottom 0.254: v6.6,12.19 v5.08,12.19
  other vias: 76.2,39.62 76.2,34.04
  pour GND: 0.76,99.06 0.76,0.76 1.27,0.25 78.49,0.25 78.99,0.76 78.99,99.06 78.49,99.57 1.27,99.57
INT
  Top 0.406: JP10.1 32.51,7.11 33.02,6.6 JTAG.2
LCDCAP_R33
  Top 0.254: U$5.6 29.54,48.94
  Top 0.406: R33.1 CLCD.1 28.79,49.7 29.54,48.94
N$1
  Top 0.254: U$5.14 22.84,44.94
  Top 0.406: 22.84,44.94 22.35,44.45 22.35,34.8 22.86,34.29 J3.2
N$2
  Top 0.254: U$5.55 39.32,56.95 38.1,58.17 38.1,63.5
  Top 0.406: 38.1,63.5 38.1,64.52 38.61,65.02 49.28,65.02 JP3.1
N$3
  Top 0.254: J8.2 R18.1
N$4
  Top 0.254: 24.64,44.45 U$5.15
  Top 0.406: TP7.1 24.38,44.2 24.64,44.45
N$5
  Top 0.254: L1.2 14.48,20.07 14.22,19.81 14.22,18.8 14.73,18.29 16,18.29 16.22,18.07 U$13.2
N$6
  Top 0.406: J7.2 43.18,16.76 43.69,16.26 R17.1
N$7
  Top 0.406: R17.2 49.65,16.26 LED1.A
N$8
  Top 0.254: LED2.A 48.3,34.9 R18.2
N$9
  Top 0.406: BATT.1 9.91,81.03 B1.+
N$10
  Top 0.406: R48.2 44.03,13.37 43.69,13.72 41.66,13.72 41.15,14.22 41.15,17.78 39.88,19.05 JP4.1
N$11
  Top 0.254: R19.1 59.18,44.2 59.69,43.69 59.69,37.34 59.49,37.14 U$1.6
N$12
  Top 0.254: JTAG.14 49.28,5.08 64.52,5.08 67.56,8.13 J6.1
N$13
  Top 0.254: U$5.49 43.74,53.29 43.94,53.09 C19.1 R44.2
N$14
  Top 0.254: U$5.54 39.82,58.87 40.22,59.27 C30.1
  Top 0.406: C30.1 40.64,59.69 40.98,60.03 U$11.3
N$15
  Top 0.254: C11.2 R11.2
N$16
  Top 0.254: U$2.6 67.11,38.55 66.55,39.12 66.55,44.2 65.28,45.47 R03.2
N$17
  Top 0.254: R08.2 69.98,47.69 U$4.5 69.98,50.42 69.85,50.55 64.6,50.55 R09.1
N$18
  Top 0.254: R13.1 69.34,52.32 69.98,52.96 U$4.4
  Top 0.406: R16.2 69.15,57.59 69.98,56.77 U$4.4
N$19
  Top 0.406: R26.1 8.38,35.05 8.76,34.67 RF1.10
N$20
  Top 0.406: RF1.12 10.03,34.67 10.67,35.31 R34.1
N$21
  Top 0.254: R15.2 71.14,58.33 R16.1
  Top 0.406: R15.2 73.66,57.66 73.79,57.53 U$4.1
N$22
  Top 0.406: C16.2 R15.1
N$23
  Top 0.406: RF1.14 11.3,33.91 12.95,35.56 R35.1
N$24
  Top 0.254: U$4.8 73.79,47.88 73.15,47.24 73.15,46.55 R08.1 73.09,43.11 72.64,42.67 71.46,42.67 R10.2
N$25
  Top 0.254: R10.1 C8.2
N$26
  Top 0.406: RF1.16 12.57,33.15 15.24,35.81 R36.1
N$27
  Top 0.406: RF1.18 13.84,32.89 17.53,36.58 R37.1
N$28
  Top 0.406: R38.1 16.85,24.47 18.29,25.91 18.29,30.73 17.53,31.5 RF1.20
N$29
  Top 0.406: RF2.18 13.84,61.94 R39.1
N$30
  Top 0.406: RF2.15 12.57,53.21 12.7,53.09 R40.2
N$31
  Top 0.406: RF2.19 15.11,53.21 14.99,53.09 14.99,52.44 R41.2
N$32  (via drill 0.6)
  Top 0.254: R05.1 v50.55,38.35 | U$4.7 72.52,50.93 72.64,51.05 | 72.64,51.05 R14.2 | 72.64,51.05 v71.88,51.82
  Bottom 0.254: v50.55,38.35 51.05,38.35 51.82,39.12 51.82,44.2 52.83,45.21 65.28,45.21 v71.88,51.82
N$33
  Top 0.254: U$3.2 63.57,29.03 64.01,29.46 R42.1
N$34
  Top 0.254: U$3.3 62.92,29.03 62.48,29.46 R43.1
N$35
  Top 0.254: U$5.16 28.19,43.94 27.94,43.69
  Top 0.406: 27.94,43.69 TP8.1
N$38
  Top 0.254: 21.63,22.48 R32.2
  Top 0.406: LED3.A 21.63,22.48
N$39
  Top 0.254: U$5.51 41.32,54.53 41.56,54.77 C18.1 41.54,55.65 Q2.P2
N$40
  Top 0.406: C29.1 50.2,61.56 JP3.2 49.02,61.72 47.06,63.68 U$11.1
N$41
  Top 0.254: U$5.52 40.82,55.19 40.39,55.63 40.39,57.91 40.6,58.13 Q2.P1
  Top 0.406: Q2.P1 42.63,58.13 43.27,58.77 C17.1
N$42
  Top 0.254: JTAG.12 45.72,13.97 46.48,14.73 59.18,14.73 59.69,15.24 J5.1
P3.0_BUTTON1
  Top 0.406: S1.1 24.13,32.01 24.38,31.75 J3.1
P3.3_LED1
  Top 0.254: U$5.25 38.82,26.2 39.37,25.65 39.37,21.34 39.62,21.08 42.93,21.08 43.18,20.83 J7.1
P3.6_LED2
  Top 0.254: U$5.28 40.32,35.63 40.89,35.05 J8.1
P3.7_R5
  Top 0.254: U$5.29 40.82,38.68 41.15,38.35 R05.2
R28
  Top 0.254: U$5.7 24.71,48.44 24.13,49.02
  Top 0.406: R28.1 R33.2 24.89,54.61 24.13,53.85 24.13,49.02
R29
  Top 0.254: U$5.8 24.19,47.94 23.37,48.77 | 23.88,57.66 28.45,57.66 | 28.7,58.84 R29.1
  Top 0.406: 23.37,48.77 23.37,57.15 23.88,57.66 | 28.7,58.84 28.7,57.91 28.45,57.66 28.79,57.32 R28.2
R30
  Top 0.254: U$5.9 23.68,47.44 22.61,48.51
  Top 0.406: 22.61,48.51 22.61,58.42 23.11,58.93 R29.2 R30.1
RESET  (via drill 0.6)
  Top 0.406: JP5.3 37.34,13.72 v37.85,13.21 | JTAG.11 46.48,3.56 46.99,4.06 v46.99,12.45 46.99,13.46 47.5,13.97 50.29,13.97 50.63,13.63 R51.2 C53.2 52.74,7.71 53.59,6.86 RESET.1
  Bottom 0.406: v37.85,13.21 46.23,13.21 v46.99,12.45
RESETCC  (via drill 0.6)
  Top 0.254: U$5.41 40.96,47.94 40.64,48.26 37.08,48.26 36.32,49.02 v35.81,49.02
  Top 0.406: R21.1 v6.1,20.57 | R40.1 v12.7,49.28 10.92,47.5 4.32,47.5 v3.3,46.48
  Bottom 0.406: v6.1,20.57 4.83,20.57 4.32,21.08 4.32,38.35 3.05,39.62 3.05,46.23 v3.3,46.48 | v12.7,49.28 12.95,49.02 v35.81,49.02
RF2_GPIO1  (via drill 0.6)
  Top 0.254: U$5.44 41.74,49.44 40.89,50.29 37.85,50.29 37.59,50.04 v37.08,50.04
  Top 0.406: R41.1 15.02,50.51 15.49,50.04 v16.76,50.04
  Bottom 0.406: v16.76,50.04 v37.08,50.04
RF2_GPIO2  (via drill 0.6)
  Top 0.254: U$5.45 42.26,49.94 41.4,50.8 36.58,50.8 36.32,51.05 v36.07,51.05
  Top 0.406: R39.2 16,61.98 16.51,62.48 v17.02,62.48
  Bottom 0.406: v36.07,51.05 18.8,51.05 18.29,51.56 18.29,61.21 v17.02,62.48
RX
  Top 0.254: U$5.26 39.32,33.83
  Top 0.406: R04.2 64.26,18.8 64.01,18.54 54.61,18.54 53.85,18.54 39.32,33.07 39.32,33.83
RX1
  Top 0.254: R01.2 65.95,26.58 63.57,24.2 U$3.7 63.57,21.61 R04.1
RX2
  Top 0.254: R01.1 67.15,29.37 | R07.1 70.51,32.83 R42.2
  Top 0.406: 67.15,29.37 R42.2
RX_OUT
  Top 0.254: R07.2 C8.1 71.36,37.26 U$2.4
S0
  Top 0.254: U$5.5 30.57,49.44 29.97,50.04 29.97,62.99 29.46,63.5 23.88,63.5 23.37,63.5 13.21,63.5 12.19,64.52 LCD1.1
S1
  Top 0.254: U$5.4 31.08,49.94 30.48,50.55 30.48,63.5 29.72,64.26 24.38,64.26 23.88,64.26 15.75,64.26 14.73,65.28 LCD1.2
S2
  Top 0.254: U$5.3 31.35,50.44 30.99,50.8 30.99,64.01 29.97,65.02 24.64,65.02 24.38,65.02 22.86,65.02 22.35,65.53 LCD1.5
S3
  Top 0.254: U$5.2 31.86,50.94 31.5,51.31 31.5,64.52 30.23,65.79 25.65,65.79 24.89,66.55 LCD1.6
S4
  Top 0.254: U$5.1 32.12,51.44 32,51.56 32,65.28 30.73,66.55 27.94,66.55 27.43,67.06 LCD1.7
S5
  Top 0.254: LCD1.9 33.02,67.82 33.02,55.63 34.82,53.83 U$5.64
S6
  Top 0.254: U$5.61 36.32,54.36 35.56,55.12 35.56,67.82 LCD1.10
S7
  Top 0.254: LCD1.13 42.67,67.56 42.16,67.06 36.83,67.06 36.07,66.29 36.07,55.37 36.82,54.62 U$5.60
S8
  Top 0.254: LCD1.14 45.21,67.06 44.7,66.55 37.34,66.55 36.58,65.79 36.58,55.63 37.32,54.88 U$5.59
S9
  Top 0.254: LCD1.15 47.75,66.55 47.24,66.04 37.59,66.04 37.08,65.53 37.08,55.88 37.82,55.14 U$5.58
S10
  Top 0.254: LCD1.17 52.83,67.56 50.8,65.53 37.85,65.53 37.59,65.28 37.59,56.13 38.32,55.41 U$5.57
S11  (via drill 0.6)
  Top 0.254: U$5.38 43.22,46.44 42.42,47.24 40.39,47.24 v40.13,47.5 | v55.37,66.8 LCD1.18
  Bottom 0.254: v40.13,47.5 40.13,61.21 44.96,66.04 54.61,66.04 v55.37,66.8
S12  (via drill 0.6)
  Top 0.254: U$5.37 42.96,45.94 42.42,46.48 v40.89,46.48 | LCD1.21 61.47,66.8 v58.17,66.8
  Bottom 0.254: v40.89,46.48 40.89,60.45 45.97,65.53 56.9,65.53 v58.17,66.8
S13  (via drill 0.6)
  Top 0.254: U$5.36 42.44,45.44 42.42,45.47 42.16,45.47 v41.91,45.72 | v64.01,66.8 LCD1.22
  Bottom 0.254: v41.91,45.72 41.91,59.94 42.42,60.45 53.59,60.45 59.94,66.8 v64.01,66.8
SFD  (via drill 0.6)
  Top 0.254: U$5.43 41.48,48.94 40.89,49.53 v39.12,49.53
  Top 0.406: R34.2 10.67,46.23 v10.92,46.48
  Bottom 0.254: v39.12,49.53 38.86,49.28
  Bottom 0.406: 38.86,49.28 38.86,47.75 38.35,47.24 11.68,47.24 v10.92,46.48
TCK  (via drill 0.6)
  Top 0.406: JP6.3 34.8,11.18 35.31,10.67 v38.86,10.67 | 42.42,11.85 R48.1 42.33,11.09 v41.91,10.67 41.91,3.81 41.66,3.56 JTAG.7
  Bottom 0.406: v38.86,10.67 v41.91,10.67
TDI
  Top 0.406: JP8.3 29.72,9.14 30.48,8.38 36.07,8.38 36.83,7.62 36.83,3.81 36.58,3.56 JTAG.3
TDO  (via drill 0.6)
  Top 0.406: JP5.1 38.35,19.81 38.61,19.56 38.61,16.26 38.35,16 27.43,16 27.18,15.75 JP9.3 v27.18,12.45 | JTAG.1 v29.46,3.56 29.21,3.81 29.21,5.59 28.96,5.84 v28.7,5.84
  Bottom 0.406: v27.18,12.45 27.18,6.1 27.43,5.84 v28.7,5.84
TEST  (via drill 0.6)
  Top 0.254: U$5.19 35.82,25.41 v35.05,24.64
  Top 0.406: JTAG.8 40.64,12.45 39.88,13.21 JP4.3 39.88,15.75 v39.62,16 39.88,16.26 JP4.2
  Bottom 0.406: v39.62,16 34.04,16 33.78,16.26 33.78,23.37 v35.05,24.64
TMS
  Top 0.406: JP7.3 32.26,9.91 32.77,9.4 38.86,9.4 39.37,8.89 39.37,3.81 39.12,3.56 JTAG.5
TX
  Top 0.254: U$5.27 39.82,34.6 39.82,34.09
  Top 0.406: R02.2 54.19,19.72 39.82,34.09
TX1
  Top 0.254: R31.2 60.54,26.58 62.92,24.2 U$3.6 62.92,21.61 R02.1
TX2
  Top 0.254: R31.1 59.34,29.37 | R50.1 55.98,32.83 R43.2
  Top 0.406: 59.34,29.37 R43.2
TXBUF
  Top 0.254: R50.2 55.12,37.76 C11.1 | C11.1 53.68,38.27 53.09,38.86 C13.1 | U$1.4 56.97,38.43 56.81,38.27 C11.1
US_DS_SEL_1
  Top 0.254: U$5.34 46.49,44.44 46.74,44.2 R19.2
US_DS_SEL_2
  Top 0.254: U$5.35 46.47,44.94 46.99,45.47 R03.1
USB_DVCC  (via drill 0.6)
  Top 0.406: L1.1 17.02,20.07 | C25.1 17.67,15.35 v17.02,16 16.72,16.3 U$13.6 | L1.1 17,19.32 v17.53,18.8 | v19.47,21.24 19.47,20.48 19.05,20.07 L1.1
  Top 0.813: J4.1 v23.62,28.96
  PWR 0.406: v17.53,18.8 17.53,16.51 v17.02,16
  PWR 0.813: v19.47,21.24 19.47,28.36 20.07,28.96 v23.62,28.96
VCC
  Top 0.406: RF2.9 8.76,52.81 C28.+ 8.46,52.51 C27.1
VOCM
  Top 0.254: U$4.2 72.52,53.72 72.9,53.34 C12.1
VREG_EN  (via drill 0.6)
  Top 0.254: U$5.46 42.78,50.44 41.66,51.56 v39.37,51.56
  Top 0.406: R20.1 4.06,19.81 v4.83,19.05 | v19.81,52.07 v19.81,42.42
  Bottom 0.406: v19.81,52.07 38.86,52.07 v39.37,51.56 | v4.83,19.05 13.97,19.05 19.81,24.89 v19.81,42.42
XDUCER1
  Top 0.254: U$1.3 60.78,38.43 61.72,39.37 J1.2 64.77,39.37 65.58,38.56 U$2.1
XDUCER2
  Top 0.254: U$1.1 60.91,37.13 61.72,36.32 J2.2 64.77,36.32 65.71,37.26 U$2.3

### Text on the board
tNames: GND | USR BUTTON | GND | USB DVCC | S | J | S=SBW | J=JTAG | INTERNAL | DVCC | EXTERNAL
tDocu: Rev 1.0B | Ultrasonic Flow Meter | X1 | X2 | Power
